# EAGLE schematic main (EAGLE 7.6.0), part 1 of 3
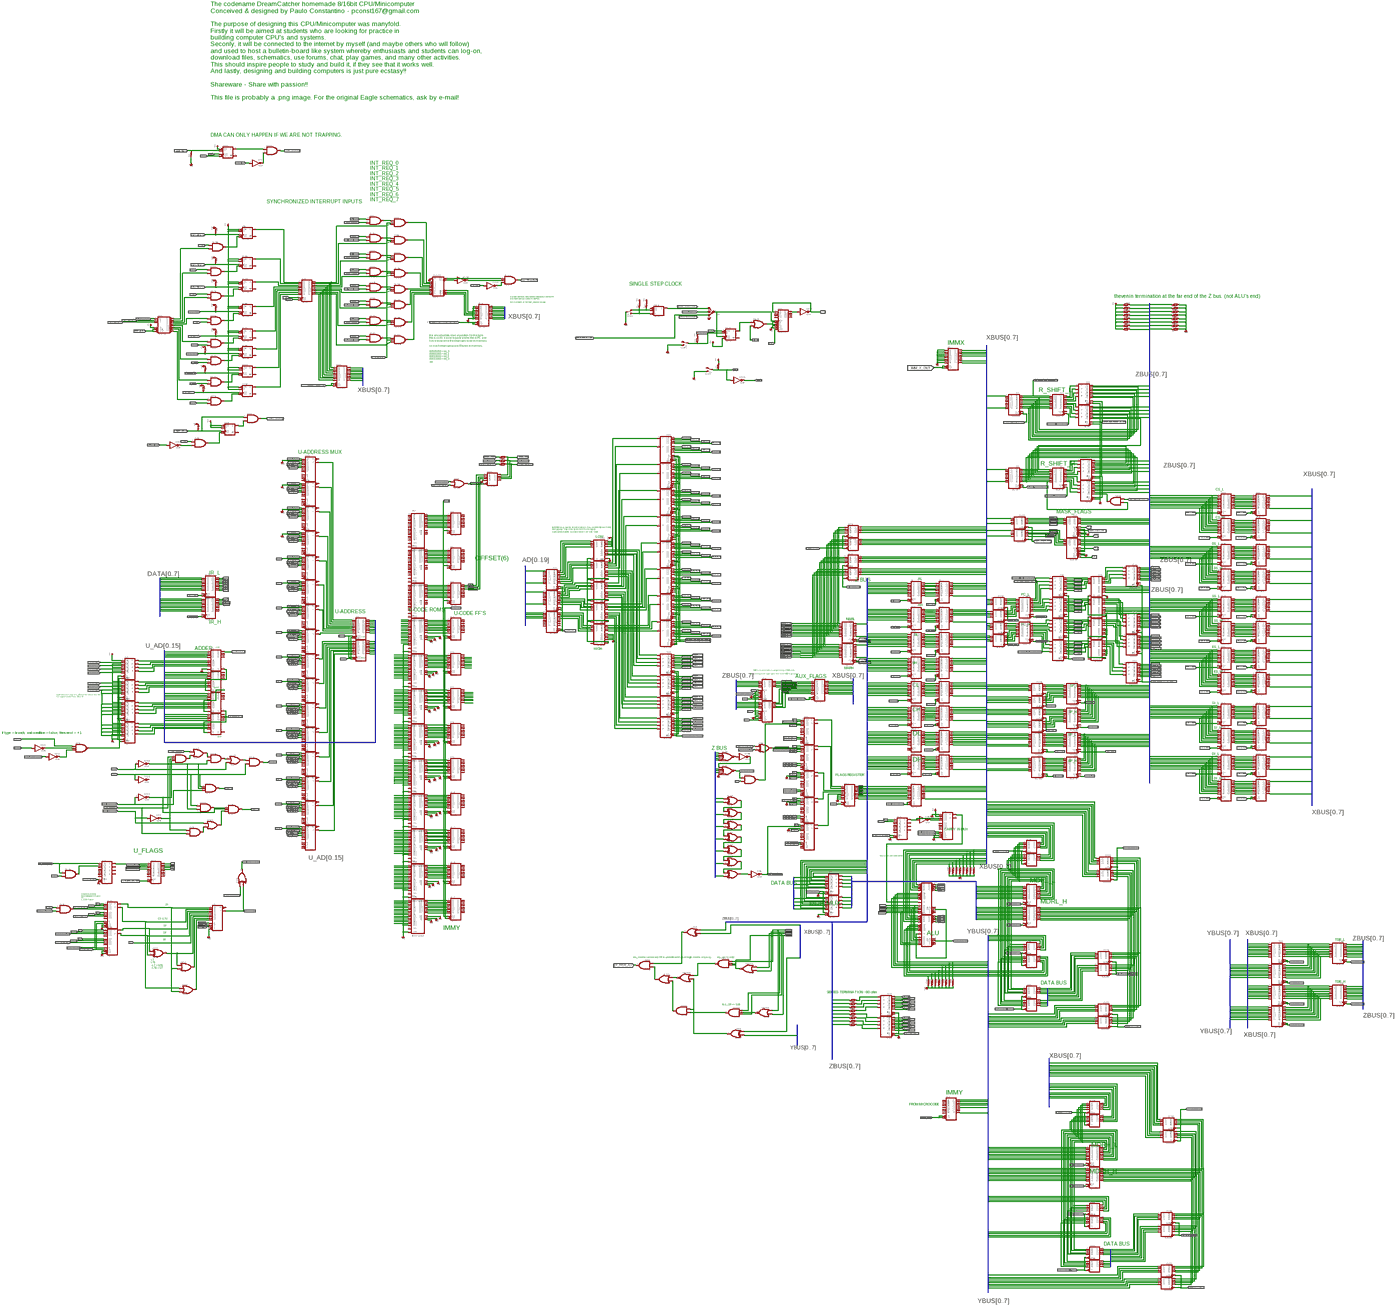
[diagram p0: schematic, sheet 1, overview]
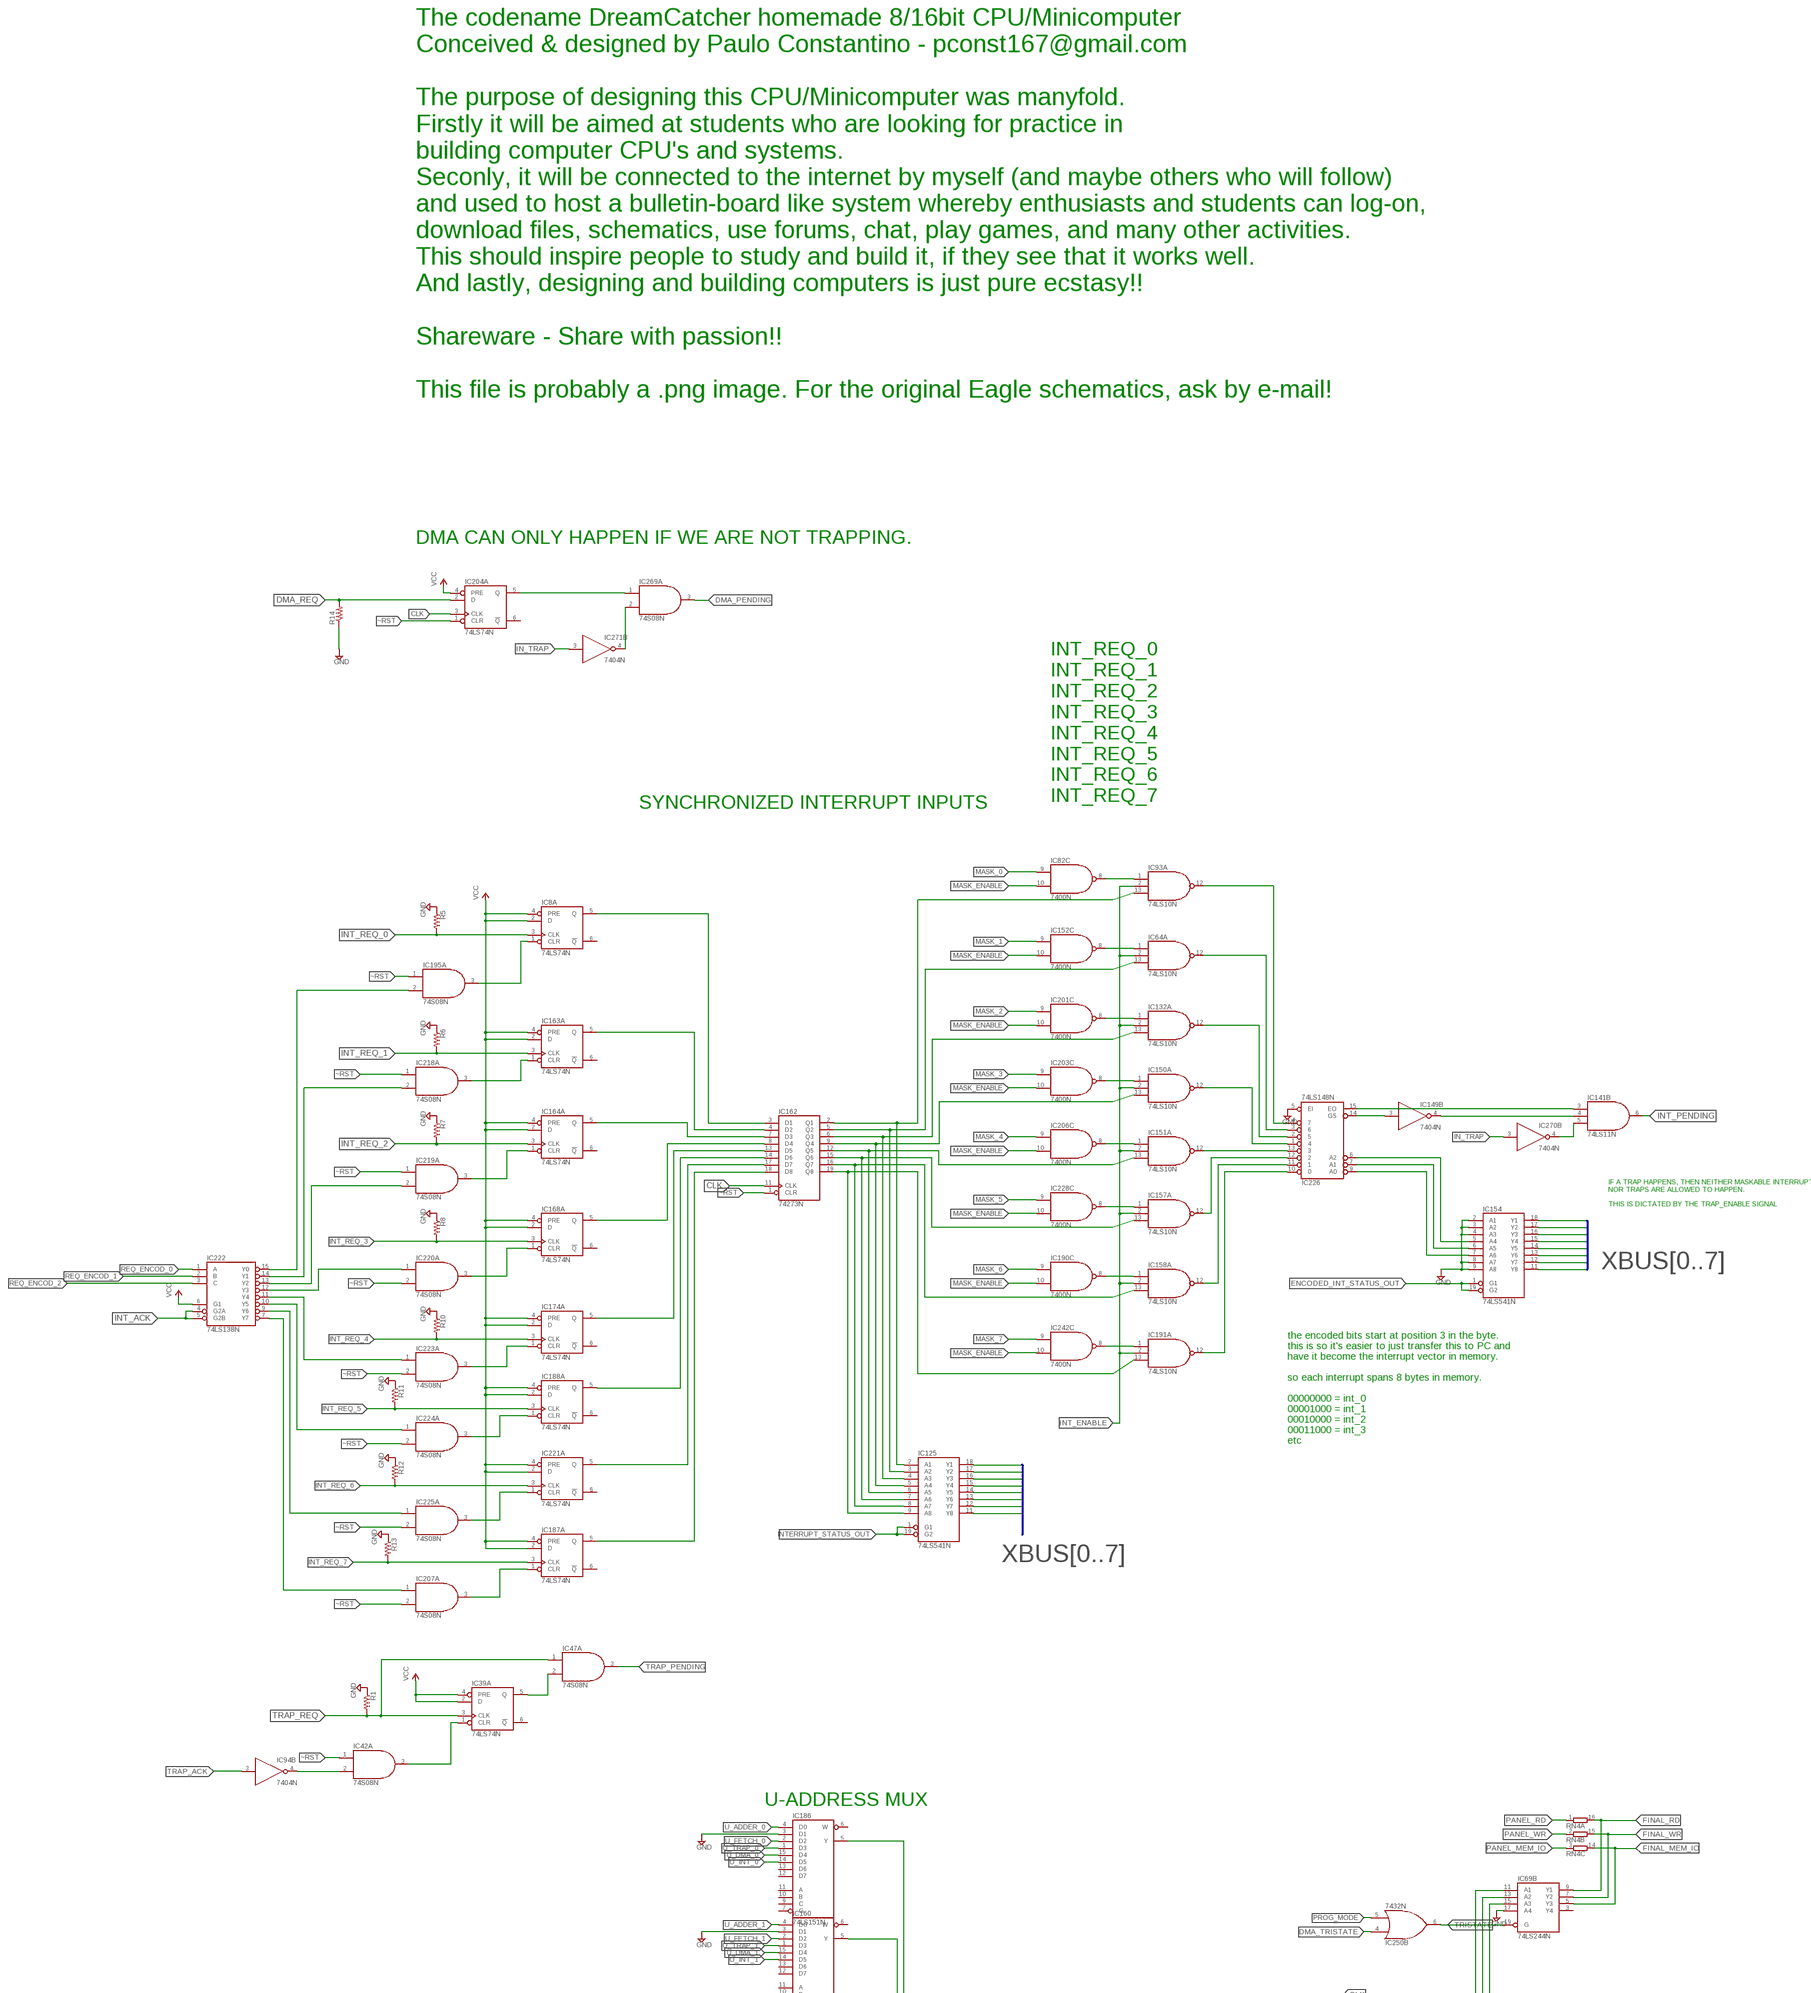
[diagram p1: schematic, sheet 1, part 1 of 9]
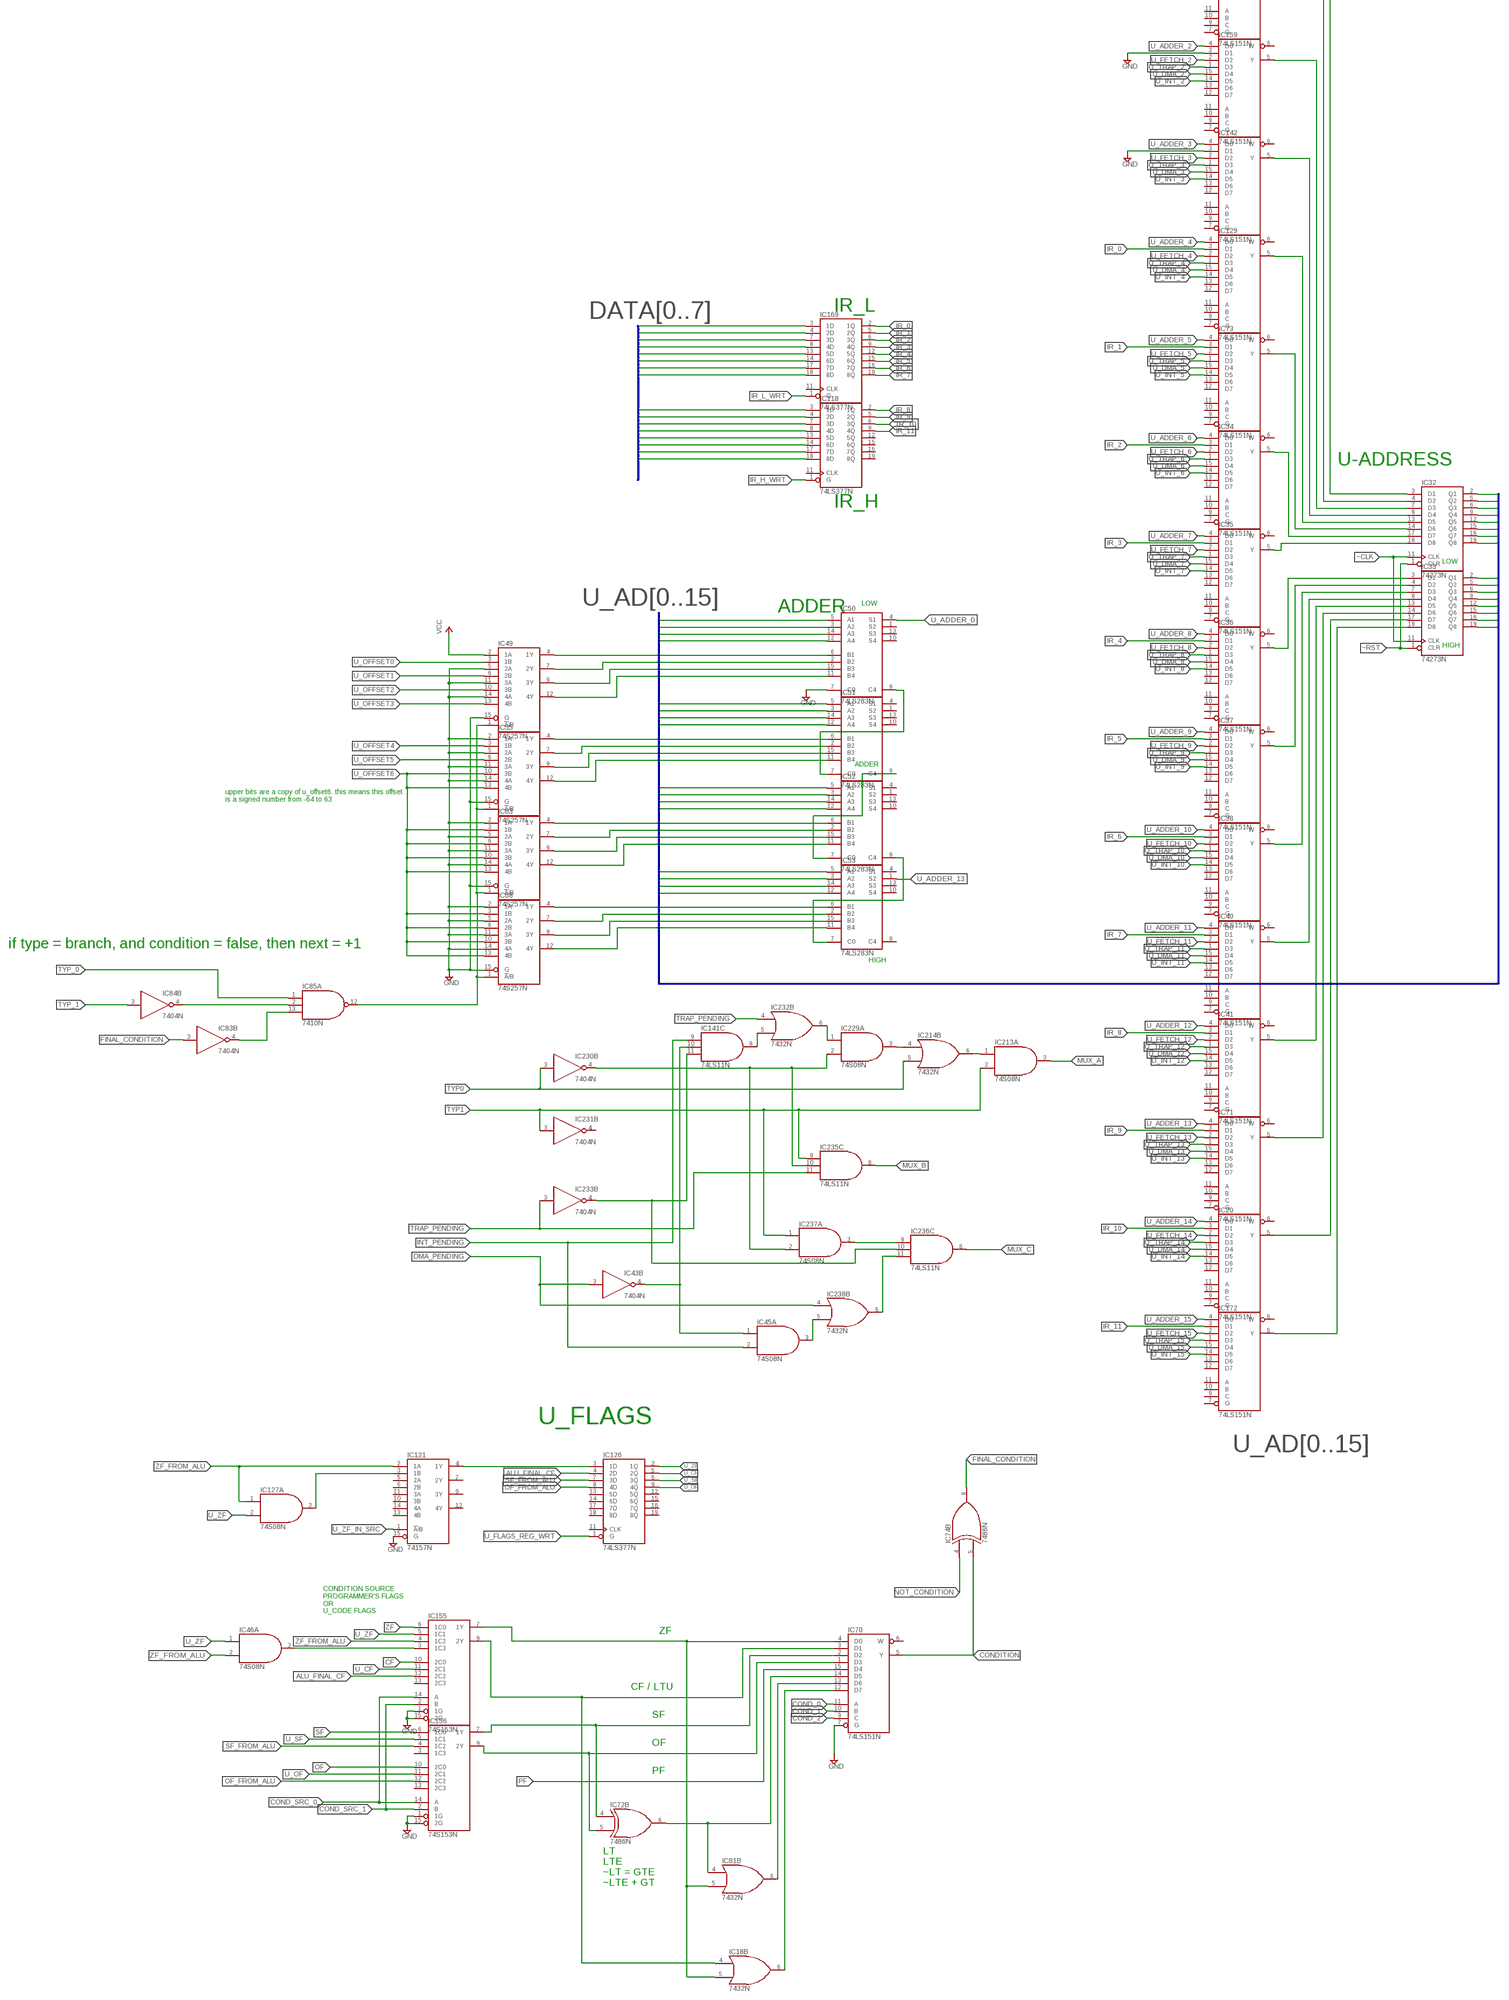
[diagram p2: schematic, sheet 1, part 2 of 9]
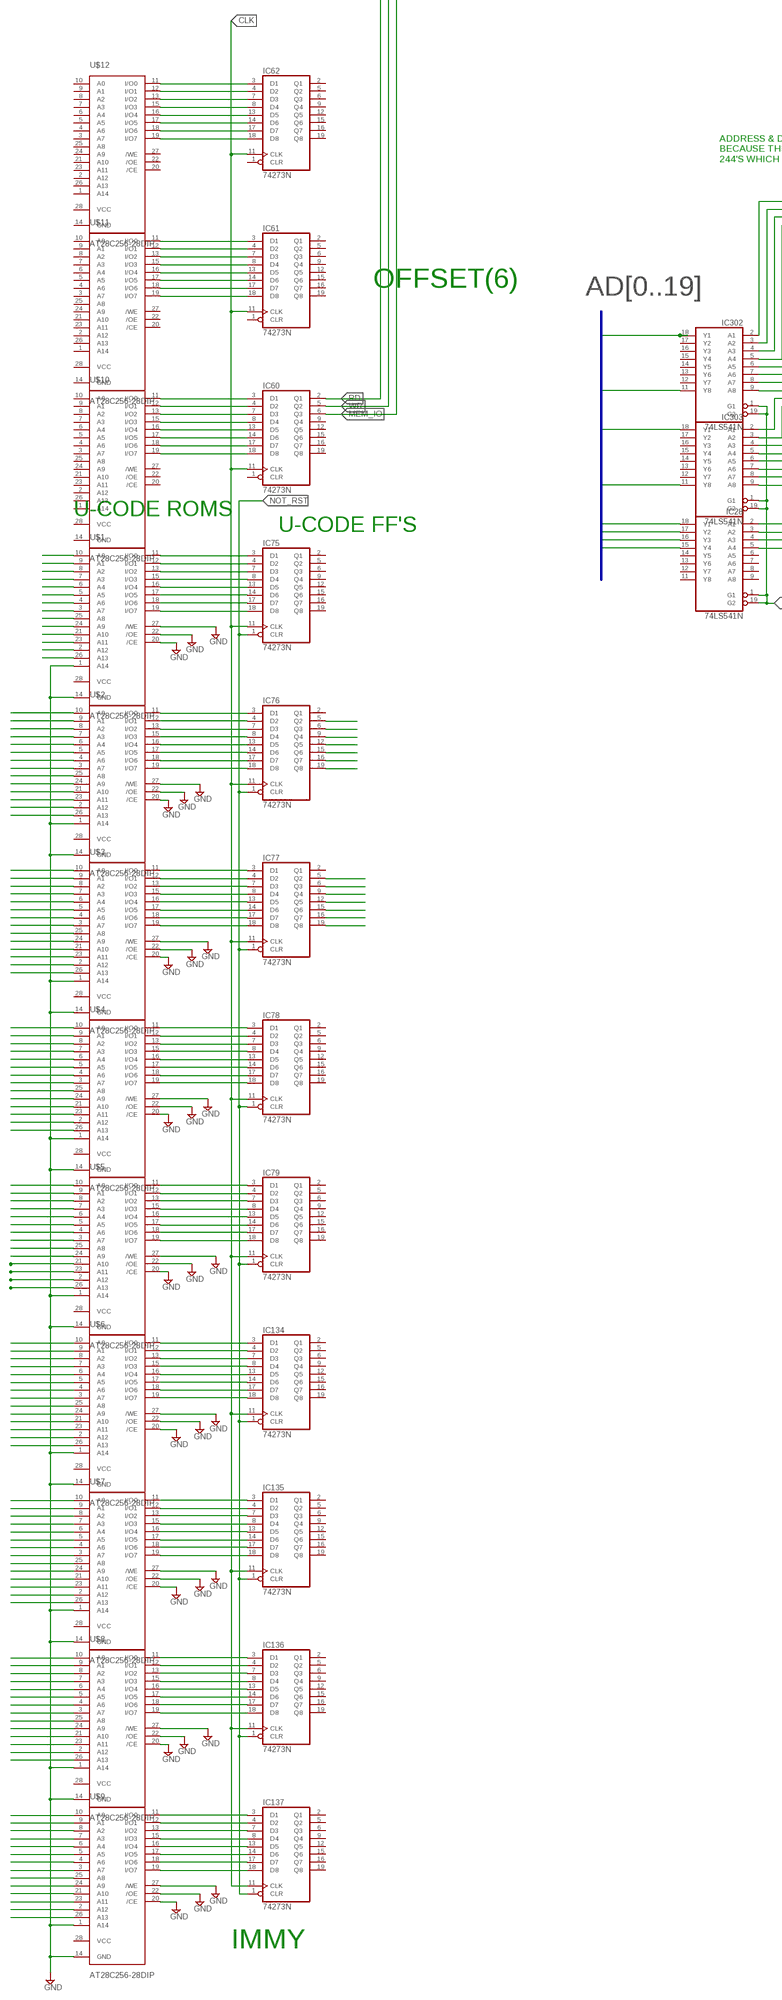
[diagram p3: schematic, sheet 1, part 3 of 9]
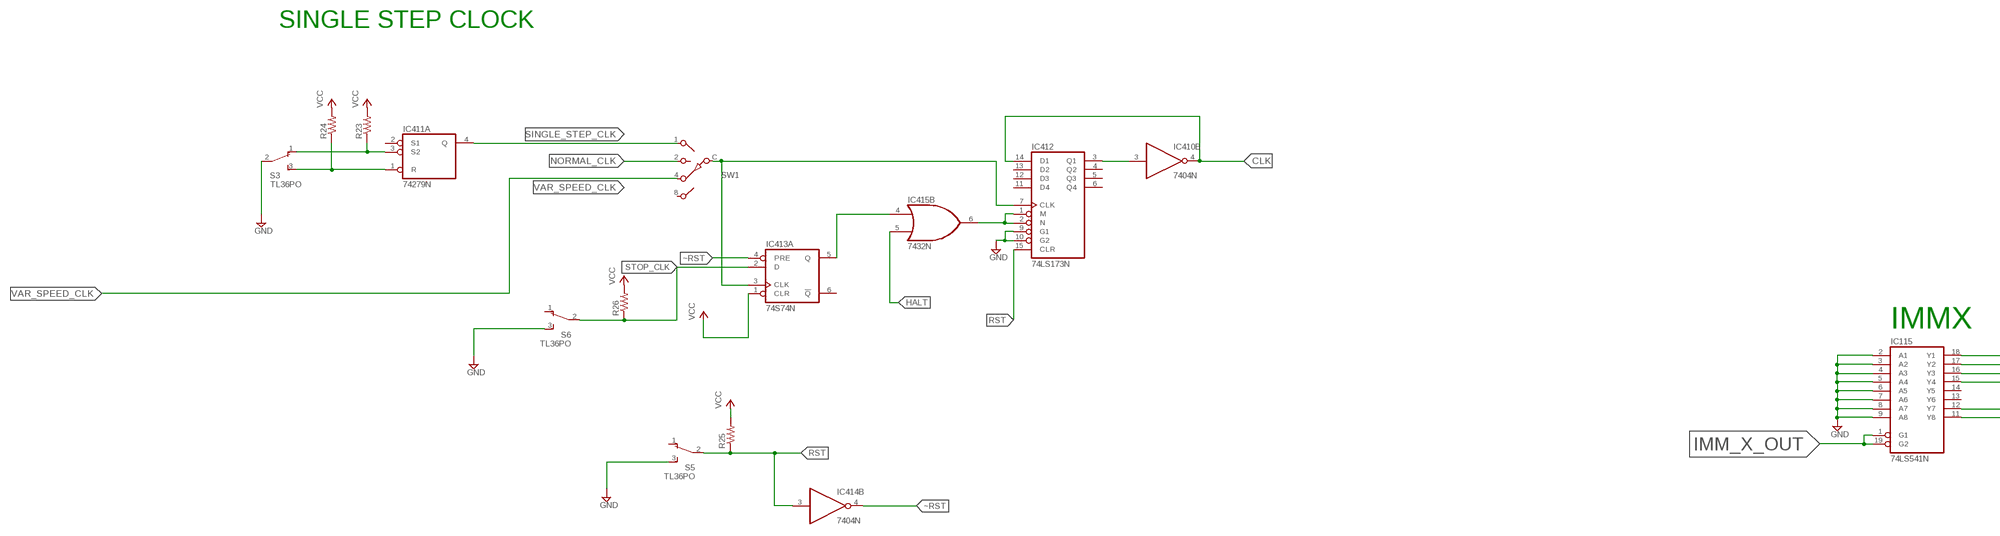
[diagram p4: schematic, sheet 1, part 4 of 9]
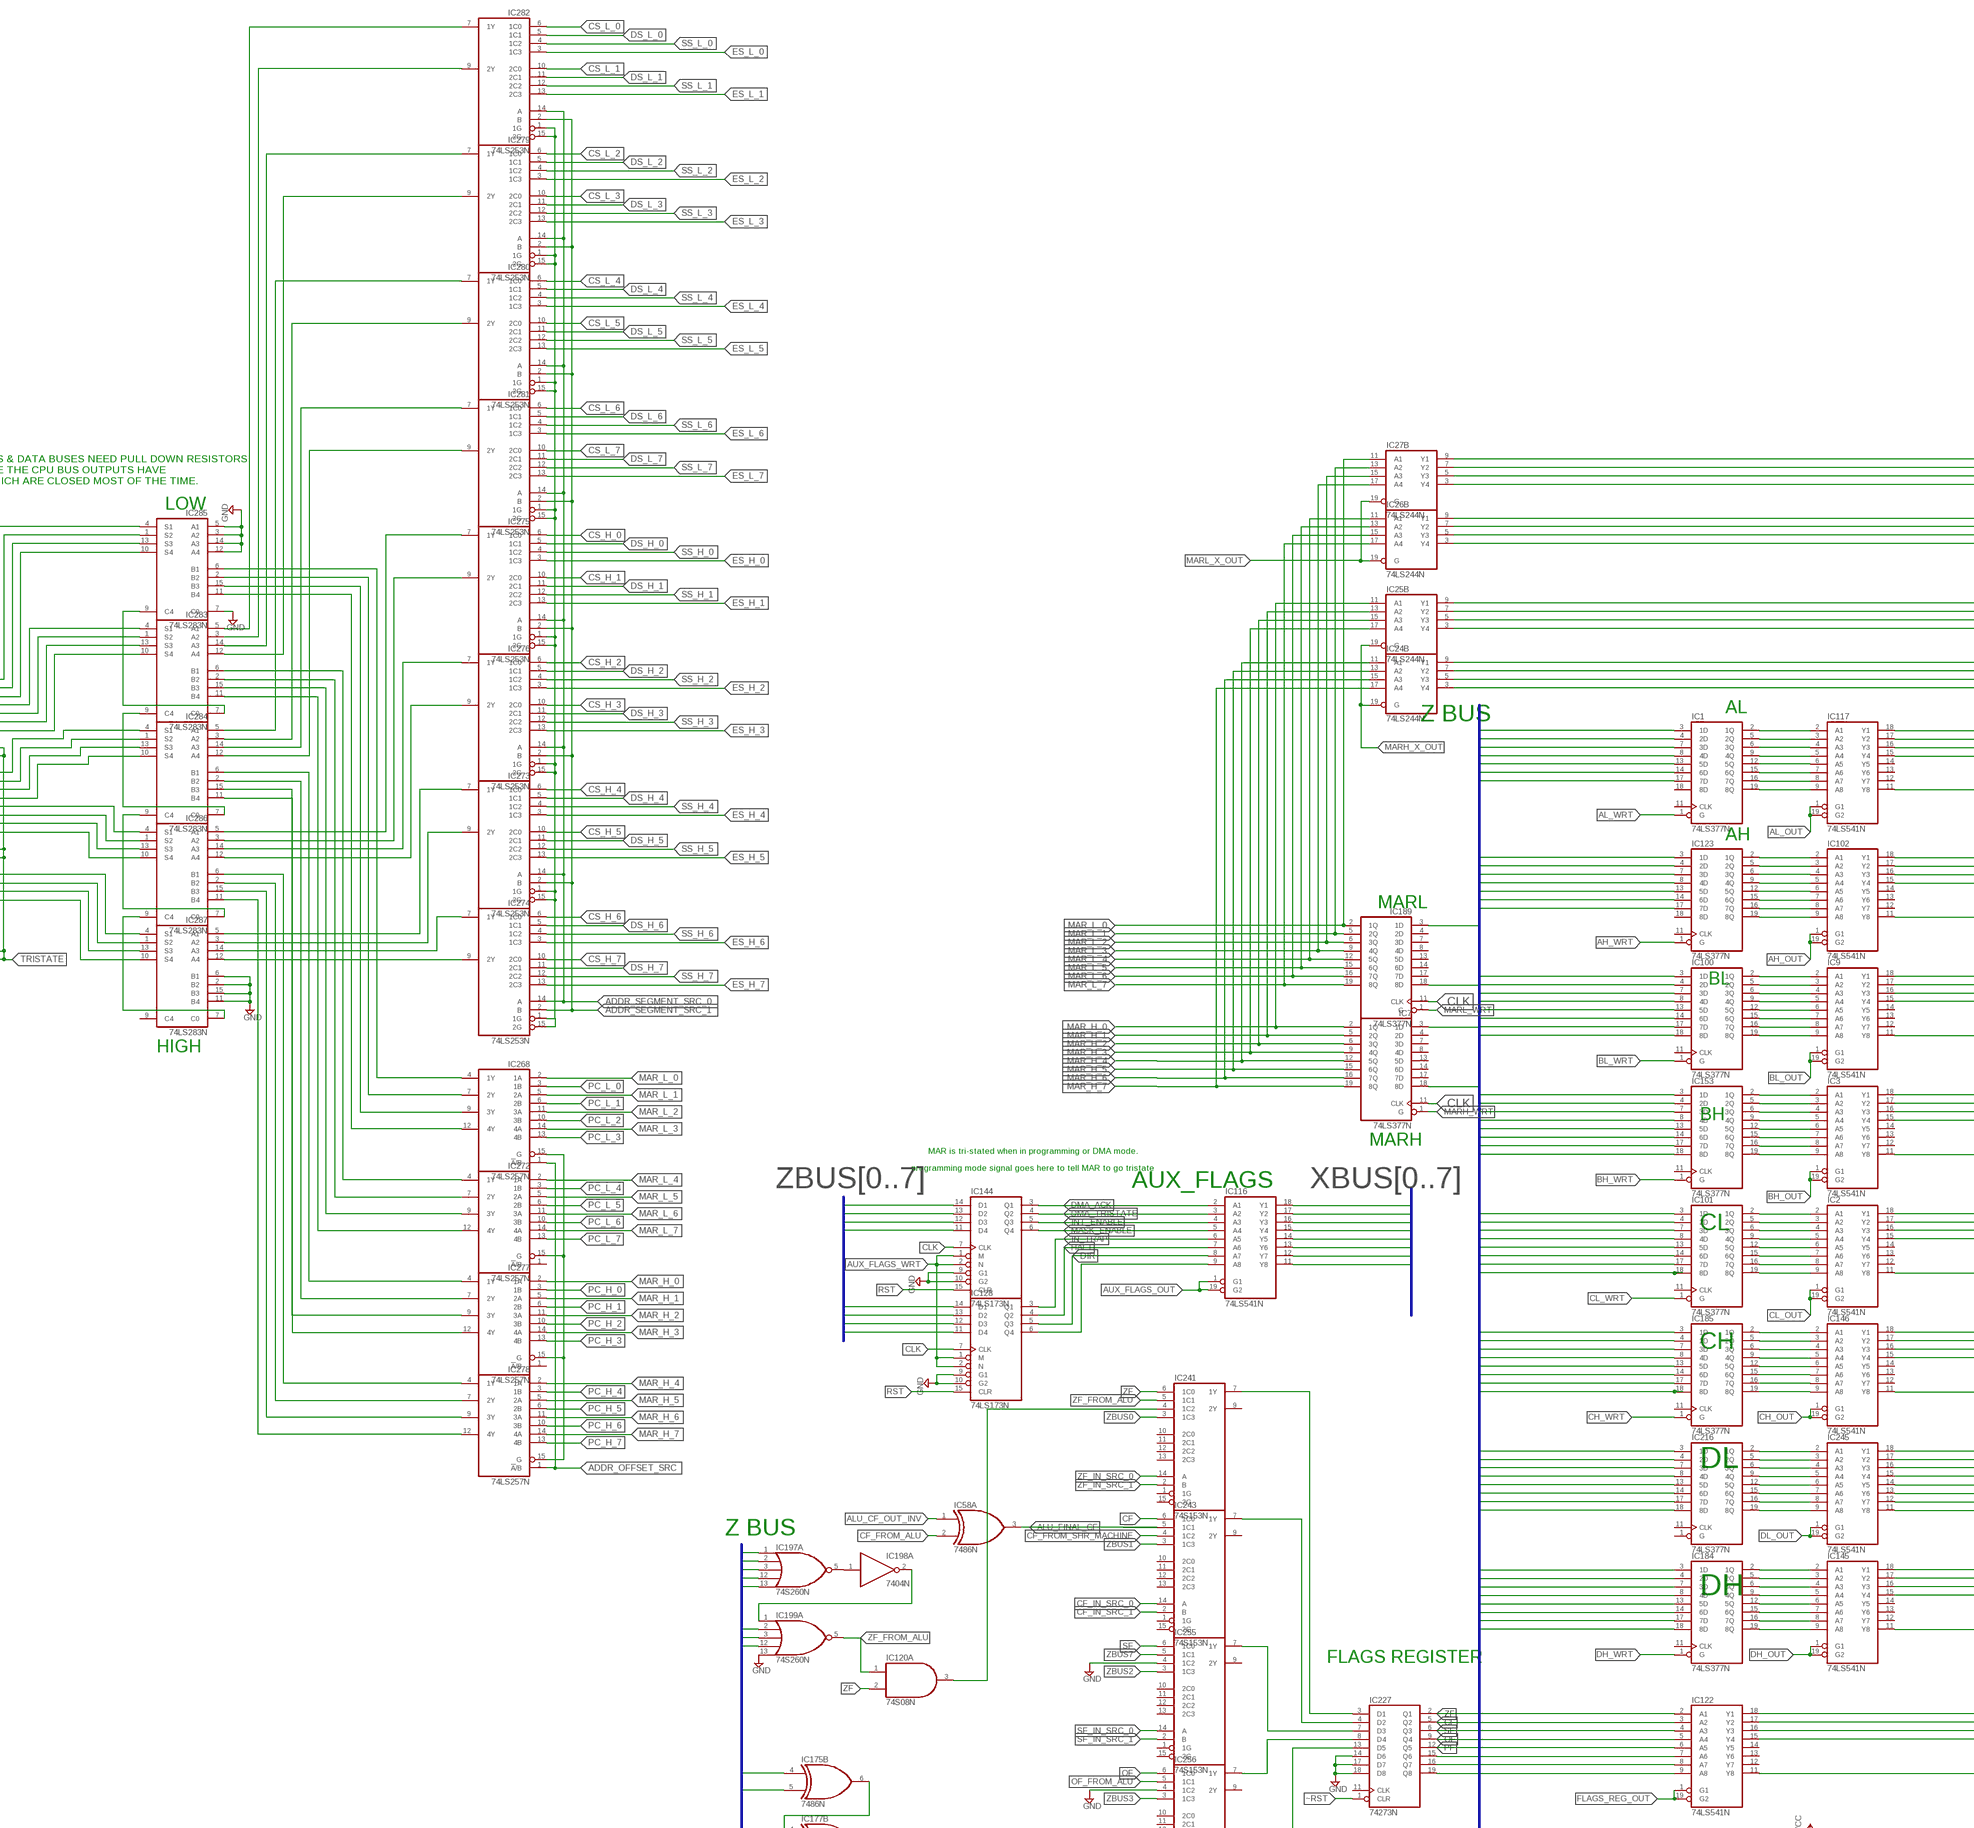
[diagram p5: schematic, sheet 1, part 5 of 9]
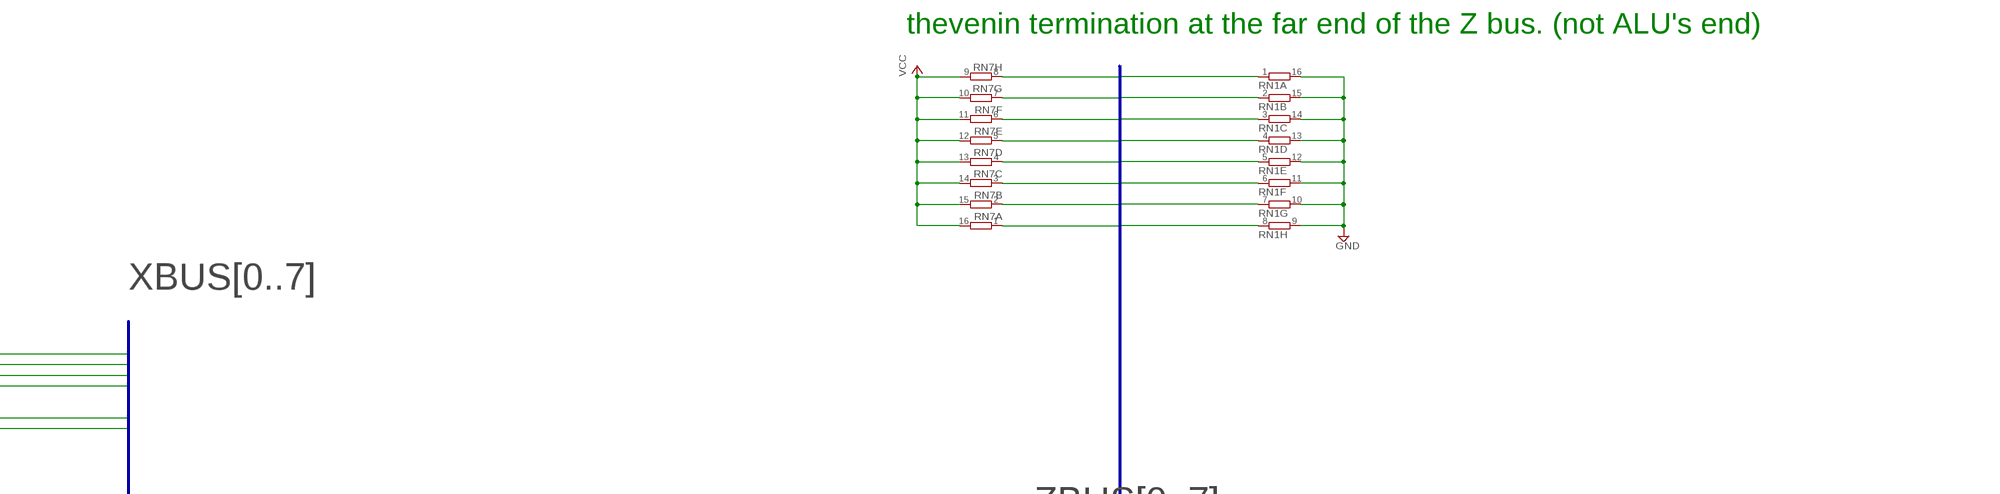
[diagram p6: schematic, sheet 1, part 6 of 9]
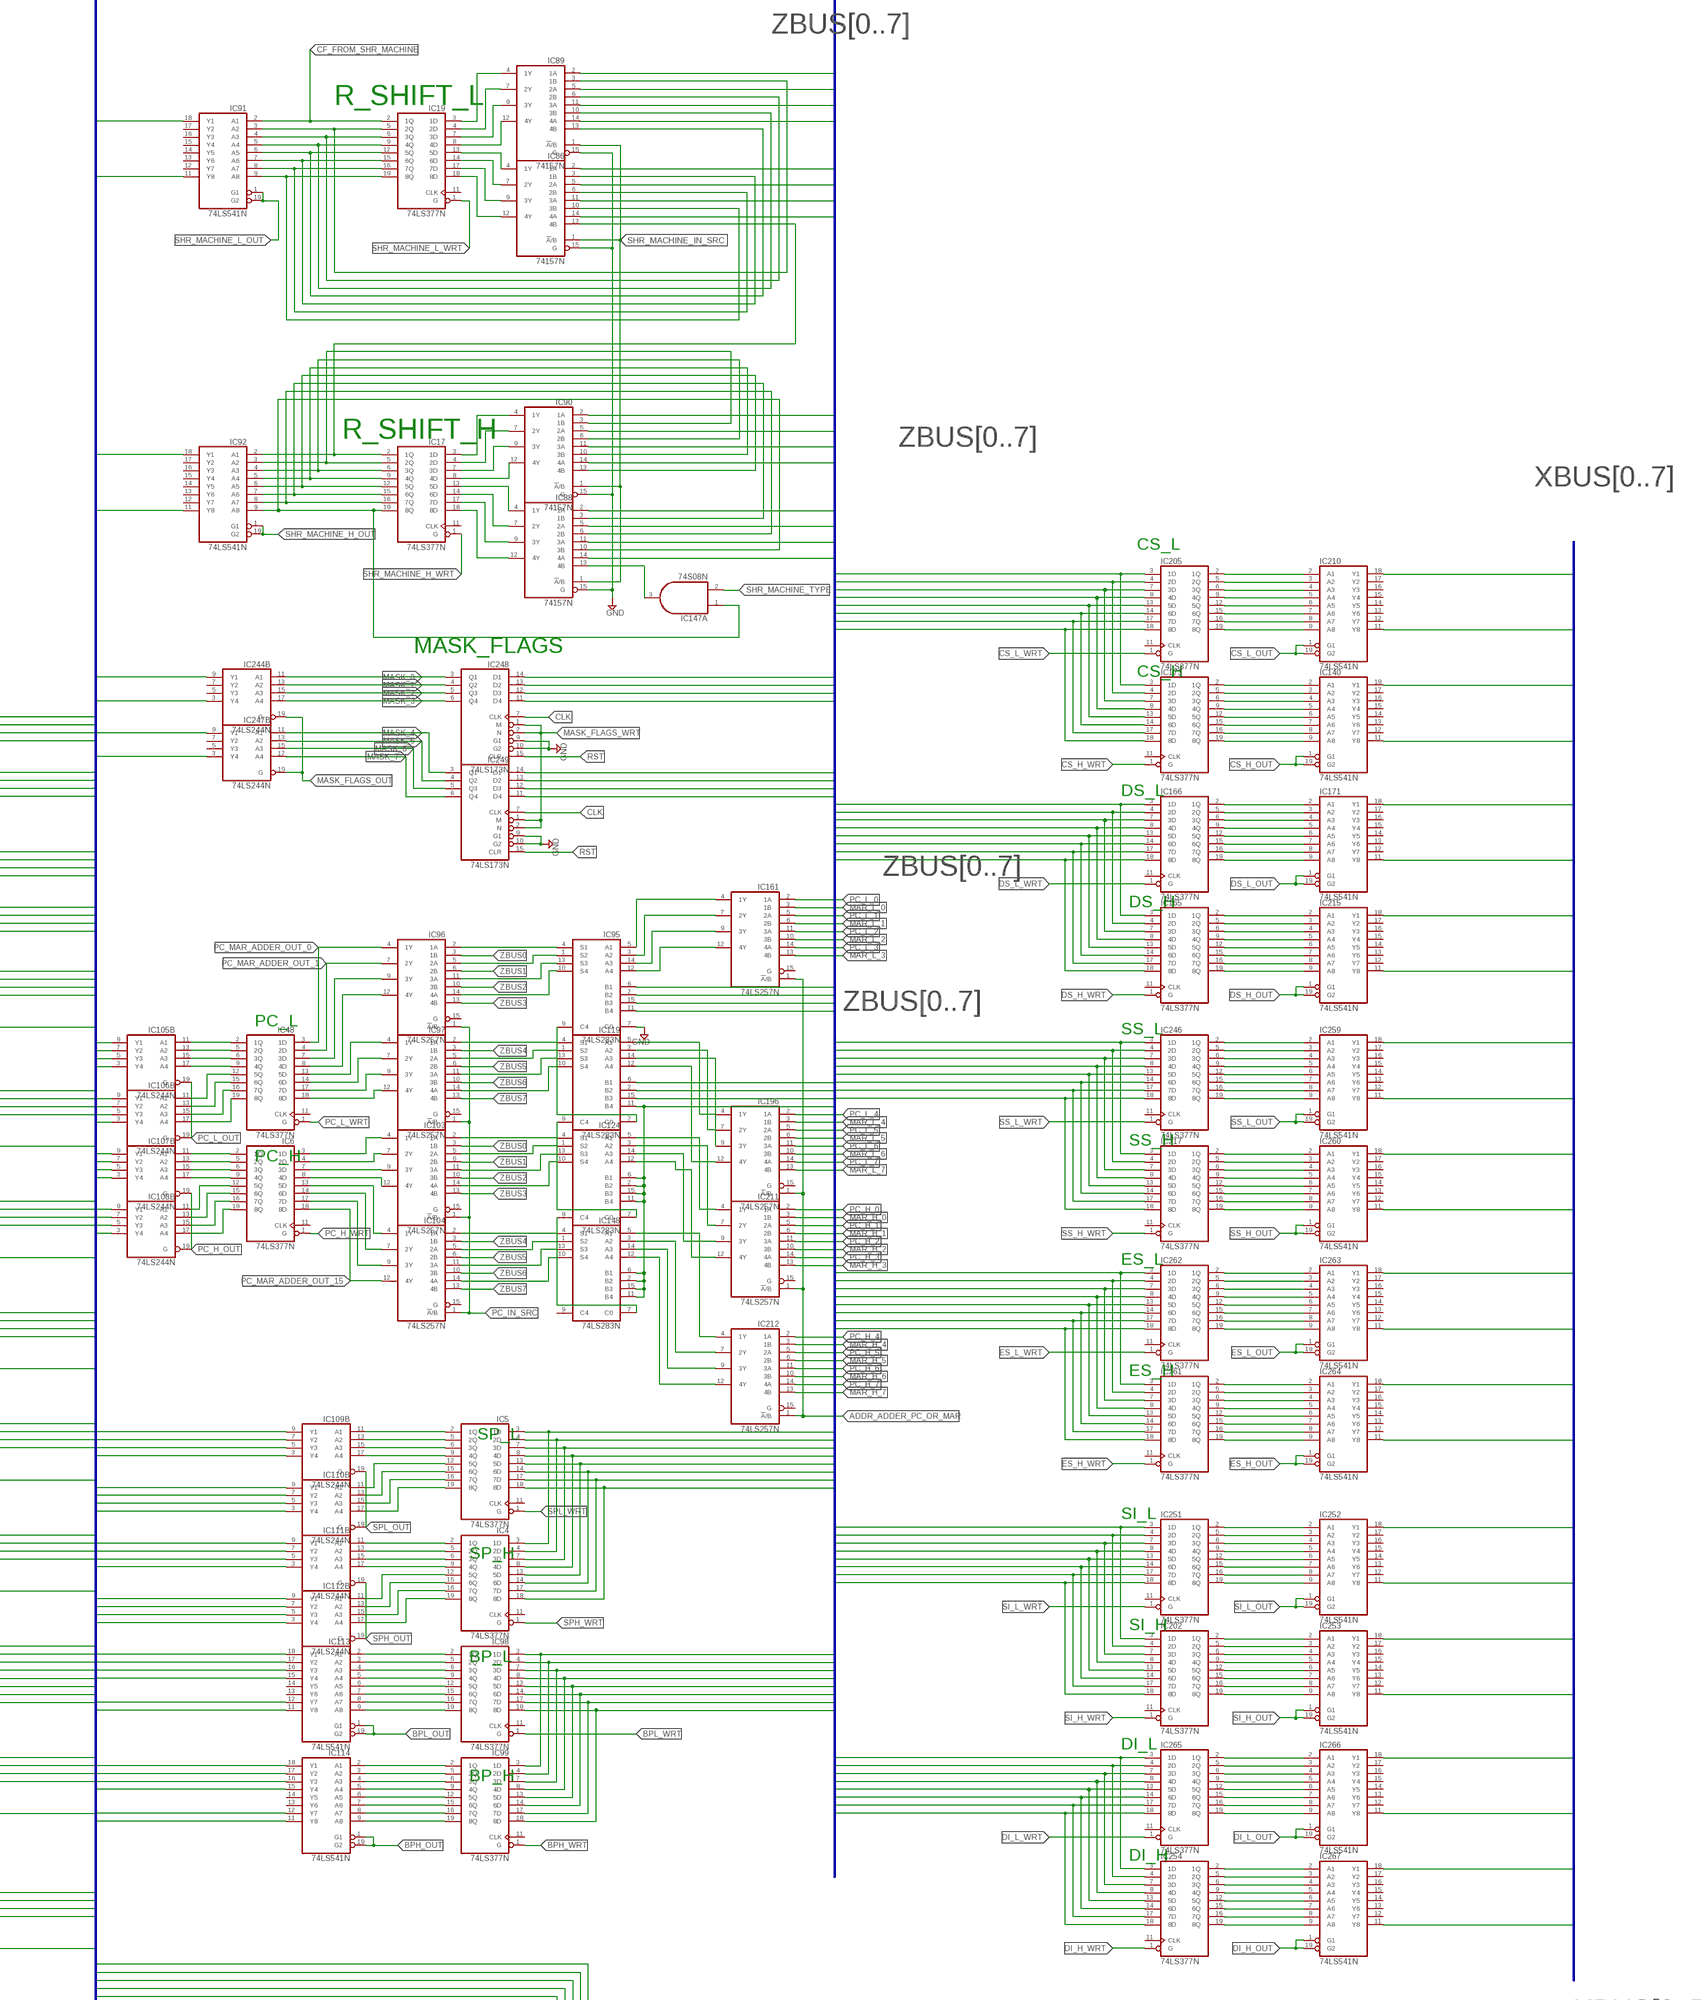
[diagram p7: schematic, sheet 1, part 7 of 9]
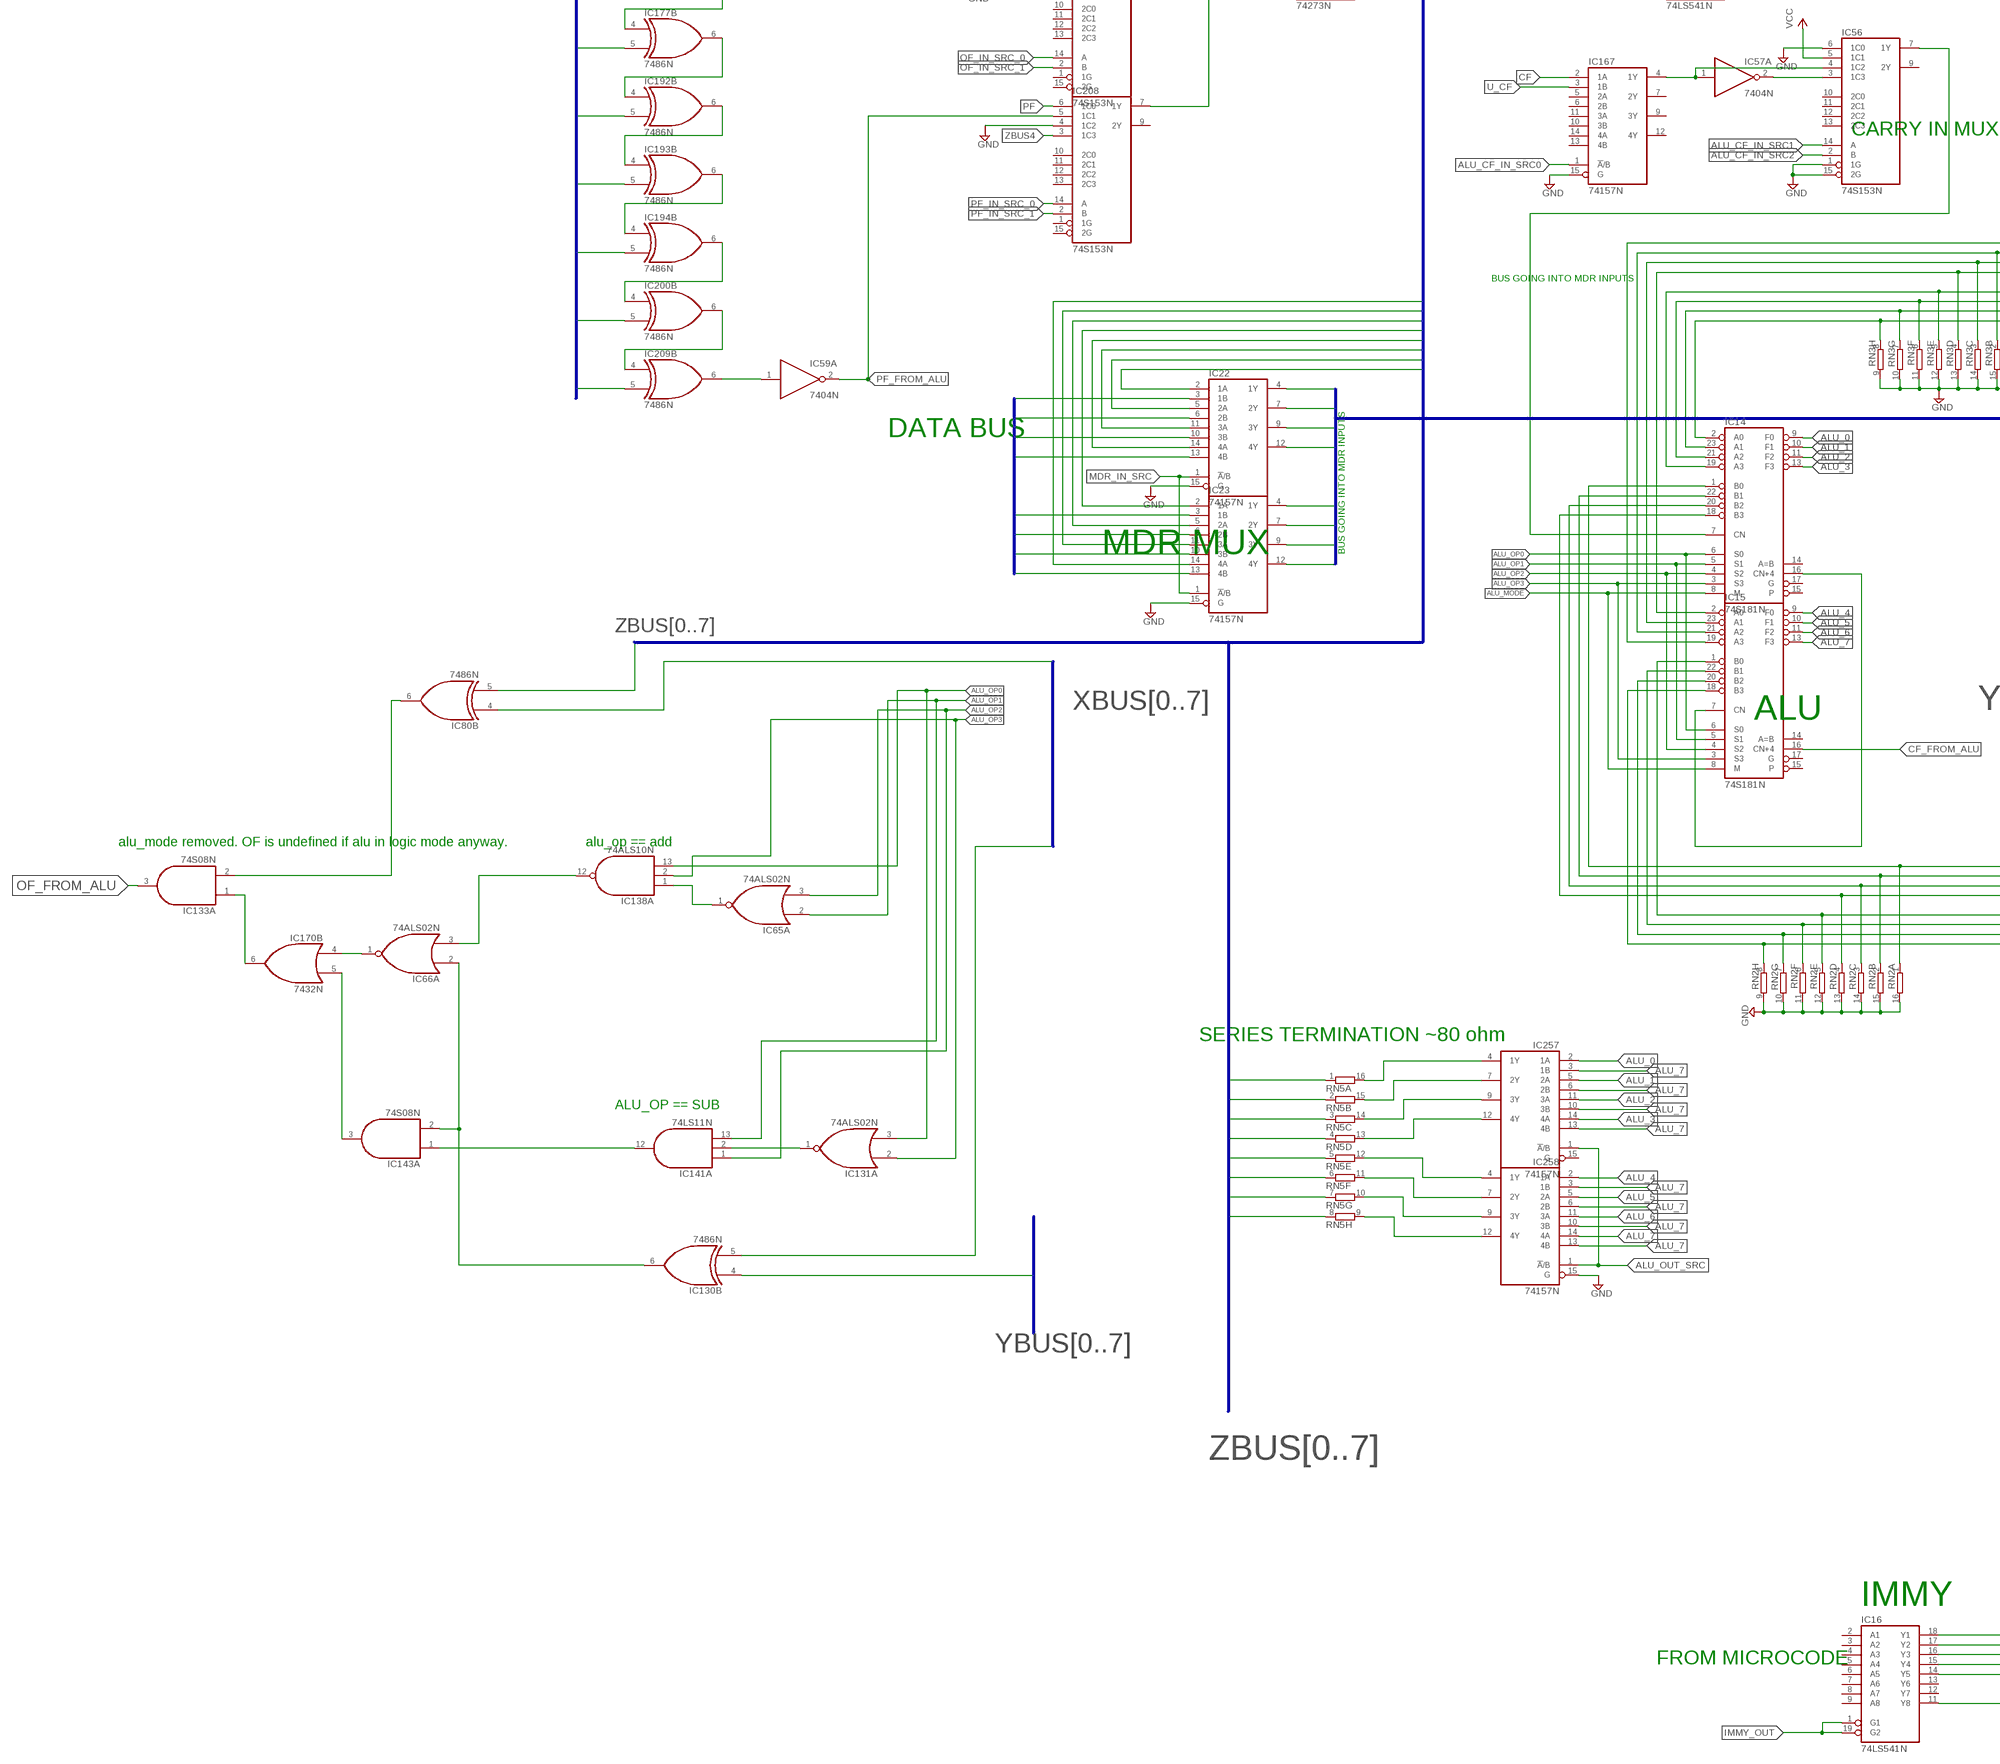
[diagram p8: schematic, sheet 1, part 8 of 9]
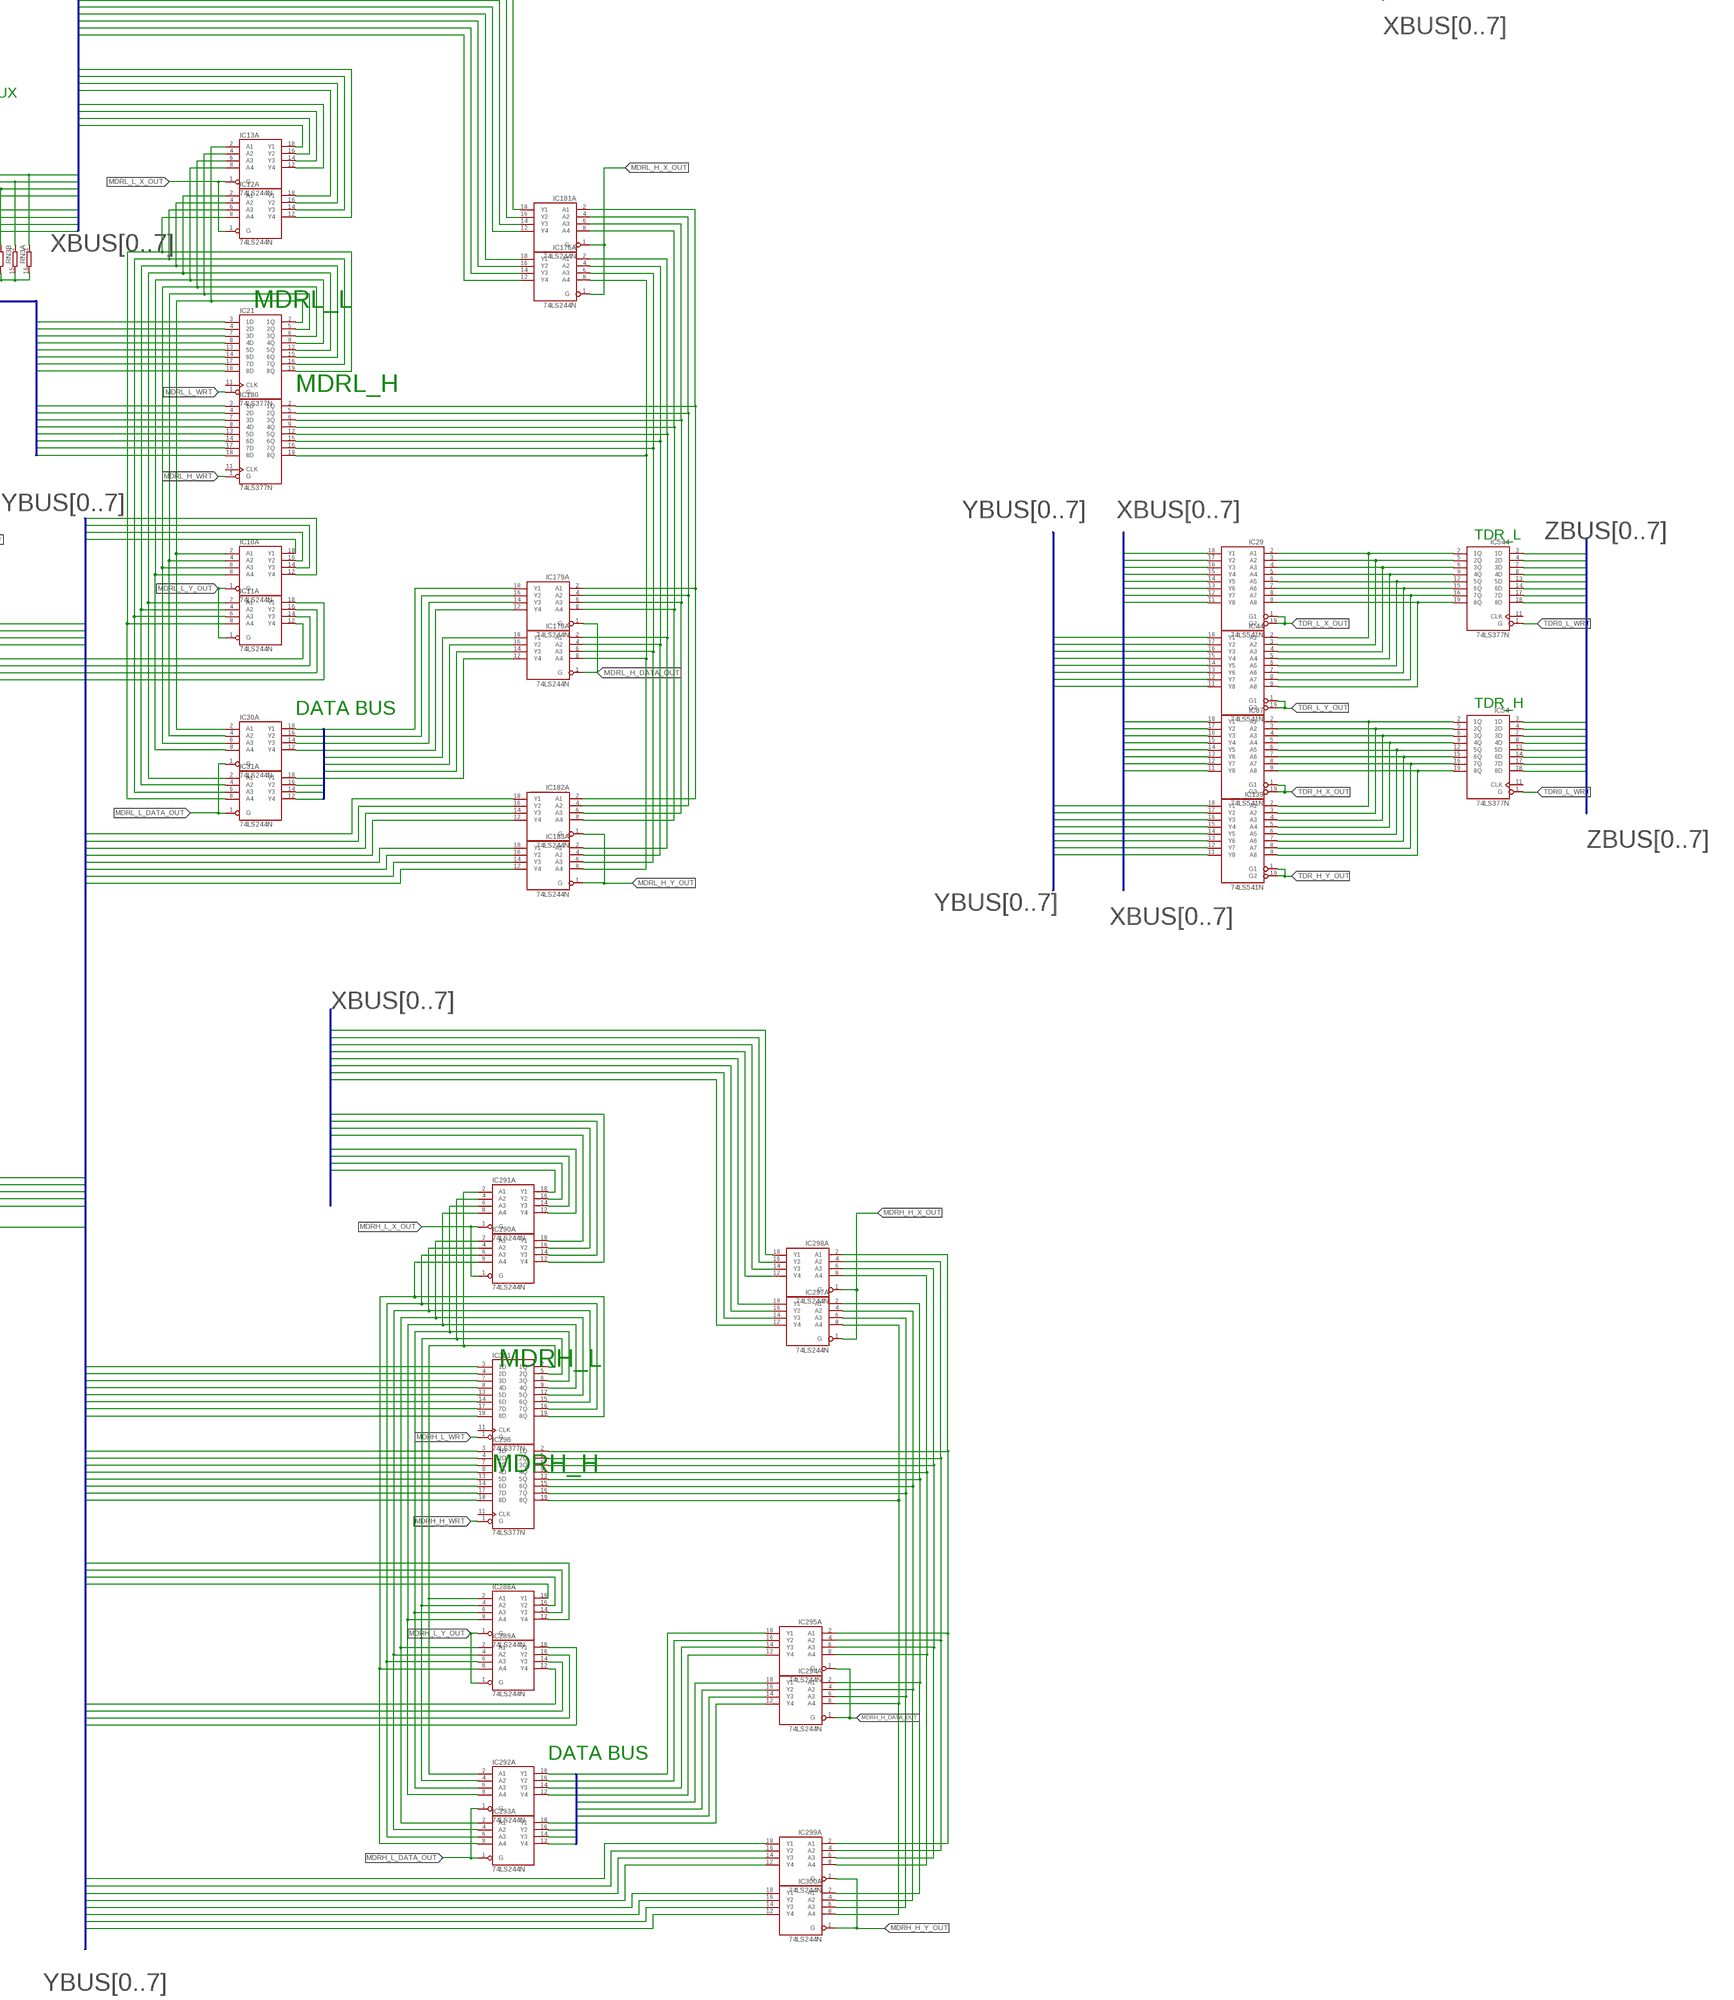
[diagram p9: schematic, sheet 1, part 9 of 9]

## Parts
IC1  74LS377N  [DIL20]
IC2  74LS541N  [DIL20]
IC3  74LS541N  [DIL20]
IC4  74LS377N  [DIL20]
IC5  74LS377N  [DIL20]
IC6  74LS377N  [DIL20]
IC7  74LS377N  [DIL20]
IC8  74LS74N  [DIL14]
IC9  74LS541N  [DIL20]
IC10  74LS244N  [DIL20]
IC11  74LS244N  [DIL20]
IC12  74LS244N  [DIL20]
IC13  74LS244N  [DIL20]
IC14  74S181N  [DIL24-6]
IC15  74S181N  [DIL24-6]
IC16  74LS541N  [DIL20]
IC17  74LS377N  [DIL20]
IC18  7432N  [DIL14]
IC19  74LS377N  [DIL20]
IC20  74LS151N  [DIL16]
IC21  74LS377N  [DIL20]
IC22  74157N  [DIL16]
IC23  74157N  [DIL16]
IC24  74LS244N  [DIL20]
IC25  74LS244N  [DIL20]
IC26  74LS244N  [DIL20]
IC27  74LS244N  [DIL20]
IC28  74LS541N  [DIL20]
IC29  74LS541N  [DIL20]
IC30  74LS244N  [DIL20]
IC31  74LS244N  [DIL20]
IC32  74273N  [DIL20]
IC33  74273N  [DIL20]
IC34  74LS151N  [DIL16]
IC35  74LS151N  [DIL16]
IC36  74LS151N  [DIL16]
IC37  74LS151N  [DIL16]
IC38  74LS151N  [DIL16]
IC39  74LS74N  [DIL14]
IC40  74LS151N  [DIL16]
IC41  74LS151N  [DIL16]
IC42  74S08N  [DIL14]
IC43  7404N  [DIL14]
IC44  74LS541N  [DIL20]
IC45  74S08N  [DIL14]
IC46  74S08N  [DIL14]
IC47  74S08N  [DIL14]
IC48  74LS377N  [DIL20]
IC49  74S257N  [DIL16]
IC50  74LS283N  [DIL16]
IC51  74LS283N  [DIL16]
IC52  74LS283N  [DIL16]
IC53  74LS283N  [DIL16]
IC54  74LS377N  [DIL20]
IC55  74S257N  [DIL16]
IC56  74S153N  [DIL16]
IC57  7404N  [DIL14]
IC58  7486N  [DIL14]
IC59  7404N  [DIL14]
IC60  74273N  [DIL20]
IC61  74273N  [DIL20]
IC62  74273N  [DIL20]
IC63  74S257N  [DIL16]
IC64  74LS10N  [DIL14]
IC65  74ALS02N  [DIL14]
IC66  74ALS02N  [DIL14]
IC68  74S257N  [DIL16]
IC69  74LS244N  [DIL20]
IC70  74LS151N  [DIL16]
IC71  74LS151N  [DIL16]
IC72  7486N  [DIL14]
IC73  74LS151N  [DIL16]
IC74  7486N  [DIL14]
IC75  74273N  [DIL20]
IC76  74273N  [DIL20]
IC77  74273N  [DIL20]
IC78  74273N  [DIL20]
IC79  74273N  [DIL20]
IC80  7486N  [DIL14]
IC81  7432N  [DIL14]
IC82  7400N  [DIL14]
IC83  7404N  [DIL14]
IC84  7404N  [DIL14]
IC85  7410N  [DIL14]
IC86  74157N  [DIL16]
IC87  74LS541N  [DIL20]
IC88  74157N  [DIL16]
IC89  74157N  [DIL16]
IC90  74157N  [DIL16]
IC91  74LS541N  [DIL20]
IC92  74LS541N  [DIL20]
IC93  74LS10N  [DIL14]
IC94  7404N  [DIL14]
IC95  74LS283N  [DIL16]
IC96  74LS257N  [DIL16]
IC97  74LS257N  [DIL16]
IC98  74LS377N  [DIL20]
IC99  74LS377N  [DIL20]
IC100  74LS377N  [DIL20]
IC101  74LS377N  [DIL20]
IC102  74LS541N  [DIL20]
IC103  74LS257N  [DIL16]
IC104  74LS257N  [DIL16]
IC105  74LS244N  [DIL20]
IC106  74LS244N  [DIL20]
IC107  74LS244N  [DIL20]
IC108  74LS244N  [DIL20]
IC109  74LS244N  [DIL20]
IC110  74LS244N  [DIL20]
IC111  74LS244N  [DIL20]
IC112  74LS244N  [DIL20]
IC113  74LS541N  [DIL20]
IC114  74LS541N  [DIL20]
IC115  74LS541N  [DIL20]
IC116  74LS541N  [DIL20]
IC117  74LS541N  [DIL20]
IC118  74LS377N  [DIL20]
IC119  74LS283N  [DIL16]
IC120  74S08N  [DIL14]
IC121  74157N  [DIL16]
IC122  74LS541N  [DIL20]
IC123  74LS377N  [DIL20]
IC124  74LS283N  [DIL16]
IC125  74LS541N  [DIL20]
IC126  74LS377N  [DIL20]
IC127  74S08N  [DIL14]
IC128  74LS173N  [DIL16]
IC129  74LS151N  [DIL16]
IC130  7486N  [DIL14]
IC131  74ALS02N  [DIL14]
IC132  74LS10N  [DIL14]
IC133  74S08N  [DIL14]
IC134  74273N  [DIL20]
IC135  74273N  [DIL20]
IC136  74273N  [DIL20]
IC137  74273N  [DIL20]
IC138  74ALS10N  [DIL14]
IC139  74LS541N  [DIL20]
IC140  74LS541N  [DIL20]
IC141  74LS11N  [DIL14]
IC142  74LS151N  [DIL16]
IC143  74S08N  [DIL14]
IC144  74LS173N  [DIL16]
IC145  74LS541N  [DIL20]
IC146  74LS541N  [DIL20]
IC147  74S08N  [DIL14]
IC148  74LS283N  [DIL16]
IC149  7404N  [DIL14]
IC150  74LS10N  [DIL14]
IC151  74LS10N  [DIL14]
IC152  7400N  [DIL14]
IC153  74LS377N  [DIL20]
IC154  74LS541N  [DIL20]
IC155  74S153N  [DIL16]
IC156  74S153N  [DIL16]
IC157  74LS10N  [DIL14]
IC158  74LS10N  [DIL14]
IC159  74LS151N  [DIL16]
IC160  74LS151N  [DIL16]
IC161  74LS257N  [DIL16]
IC162  74273N  [DIL20]
IC163  74LS74N  [DIL14]
IC164  74LS74N  [DIL14]
IC165  74LS377N  [DIL20]
IC166  74LS377N  [DIL20]
IC167  74157N  [DIL16]
IC168  74LS74N  [DIL14]
IC169  74LS377N  [DIL20]
IC170  7432N  [DIL14]
IC171  74LS541N  [DIL20]
IC172  74LS151N  [DIL16]
IC173  74LS377N  [DIL20]
IC174  74LS74N  [DIL14]
IC175  7486N  [DIL14]
IC176  74LS244N  [DIL20]
IC177  7486N  [DIL14]
IC178  74LS244N  [DIL20]
IC179  74LS244N  [DIL20]
IC180  74LS377N  [DIL20]
IC181  74LS244N  [DIL20]
IC182  74LS244N  [DIL20]
IC183  74LS244N  [DIL20]
IC184  74LS377N  [DIL20]
IC185  74LS377N  [DIL20]
IC186  74LS151N  [DIL16]
IC187  74LS74N  [DIL14]
IC188  74LS74N  [DIL14]
IC189  74LS377N  [DIL20]
IC190  7400N  [DIL14]
IC191  74LS10N  [DIL14]
IC192  7486N  [DIL14]
IC193  7486N  [DIL14]
IC194  7486N  [DIL14]
IC195  74S08N  [DIL14]
IC196  74LS257N  [DIL16]
IC197  74S260N  [DIL14]
IC198  7404N  [DIL14]
IC199  74S260N  [DIL14]
IC200  7486N  [DIL14]
IC201  7400N  [DIL14]
IC202  74LS377N  [DIL20]
IC203  7400N  [DIL14]
IC204  74LS74N  [DIL14]
IC205  74LS377N  [DIL20]
IC206  7400N  [DIL14]
IC207  74S08N  [DIL14]
IC208  74S153N  [DIL16]
IC209  7486N  [DIL14]
IC210  74LS541N  [DIL20]
IC211  74LS257N  [DIL16]
IC212  74LS257N  [DIL16]
IC213  74S08N  [DIL14]
IC214  7432N  [DIL14]
IC215  74LS541N  [DIL20]
IC216  74LS377N  [DIL20]
IC217  74LS377N  [DIL20]
IC218  74S08N  [DIL14]
IC219  74S08N  [DIL14]
IC220  74S08N  [DIL14]
IC221  74LS74N  [DIL14]
IC222  74LS138N  [DIL16]
IC223  74S08N  [DIL14]
IC224  74S08N  [DIL14]
IC225  74S08N  [DIL14]
IC226  74LS148N  [DIL16]
IC227  74273N  [DIL20]
IC228  7400N  [DIL14]
IC229  74S08N  [DIL14]
IC230  7404N  [DIL14]
IC231  7404N  [DIL14]
IC232  7432N  [DIL14]
IC233  7404N  [DIL14]
IC235  74LS11N  [DIL14]
IC236  74LS11N  [DIL14]
IC237  74S08N  [DIL14]
IC238  7432N  [DIL14]
IC241  74S153N  [DIL16]
IC242  7400N  [DIL14]
IC243  74S153N  [DIL16]
IC244  74LS244N  [DIL20]
IC245  74LS541N  [DIL20]
IC246  74LS377N  [DIL20]
IC247  74LS244N  [DIL20]
IC248  74LS173N  [DIL16]
IC249  74LS173N  [DIL16]
IC250  7432N  [DIL14]
IC251  74LS377N  [DIL20]
IC252  74LS541N  [DIL20]
IC253  74LS541N  [DIL20]
IC254  74LS377N  [DIL20]
IC255  74S153N  [DIL16]
IC256  74S153N  [DIL16]
IC257  74157N  [DIL16]
IC258  74157N  [DIL16]
IC259  74LS541N  [DIL20]
IC260  74LS541N  [DIL20]
IC261  74LS377N  [DIL20]
IC262  74LS377N  [DIL20]
IC263  74LS541N  [DIL20]
IC264  74LS541N  [DIL20]
IC265  74LS377N  [DIL20]
IC266  74LS541N  [DIL20]
IC267  74LS541N  [DIL20]
IC268  74LS257N  [DIL16]
IC269  74S08N  [DIL14]
IC270  7404N  [DIL14]
IC271  7404N  [DIL14]
IC272  74LS257N  [DIL16]
IC273  74LS253N  [DIL16]
IC274  74LS253N  [DIL16]
IC275  74LS253N  [DIL16]
IC276  74LS253N  [DIL16]
IC277  74LS257N  [DIL16]
IC278  74LS257N  [DIL16]
IC279  74LS253N  [DIL16]
IC280  74LS253N  [DIL16]
IC281  74LS253N  [DIL16]
IC282  74LS253N  [DIL16]
IC283  74LS283N  [DIL16]
IC284  74LS283N  [DIL16]
IC285  74LS283N  [DIL16]
IC286  74LS283N  [DIL16]
IC287  74LS283N  [DIL16]
IC288  74LS244N  [DIL20]
IC289  74LS244N  [DIL20]
IC290  74LS244N  [DIL20]
IC291  74LS244N  [DIL20]
IC292  74LS244N  [DIL20]
IC293  74LS244N  [DIL20]
IC294  74LS244N  [DIL20]
IC295  74LS244N  [DIL20]
IC296  74LS377N  [DIL20]
IC297  74LS244N  [DIL20]
IC298  74LS244N  [DIL20]
IC299  74LS244N  [DIL20]
IC300  74LS244N  [DIL20]
IC301  74LS377N  [DIL20]
IC302  74LS541N  [DIL20]
IC303  74LS541N  [DIL20]
IC410  7404N  [DIL14]
IC411  74279N  [DIL16]
IC412  74LS173N  [DIL16]
IC413  74S74N  [DIL14]
IC414  7404N  [DIL14]
IC415  7432N  [DIL14]
IC544  74LS377N  [DIL20]
R1  R-US_0204/7  [0204/7]
R5  R-US_0204/7  [0204/7]
R6  R-US_0204/7  [0204/7]
R7  R-US_0204/7  [0204/7]
R8  R-US_0204/7  [0204/7]
R10  R-US_0204/7  [0204/7]
R11  R-US_0204/7  [0204/7]
R12  R-US_0204/7  [0204/7]
R13  R-US_0204/7  [0204/7]
R14  R-US_0204/7  [0204/7]
R23  R-US_0204/2V  [0204V]
R24  R-US_0204/2V  [0204V]
R25  R-US_0204/2V  [0204V]
R26  R-US_0204/2V  [0204V]
RN1  8R-N  [DIL16]
RN2  8R-N  [DIL16]
RN3  8R-N  [DIL16]
RN4  8R-N  [DIL16]
RN5  8R-N  [DIL16]
RN7  8R-N  [DIL16]
S3  TL36PO  [TL3XPO]
S5  TL36PO  [TL3XPO]
S6  TL36PO  [TL3XPO]
SW1  SW-C10  [SW-C10]
U$1  AT28C256-28DIP  [DIL28-6]
U$2  AT28C256-28DIP  [DIL28-6]
U$3  AT28C256-28DIP  [DIL28-6]
U$4  AT28C256-28DIP  [DIL28-6]
U$5  AT28C256-28DIP  [DIL28-6]
U$6  AT28C256-28DIP  [DIL28-6]
U$7  AT28C256-28DIP  [DIL28-6]
U$8  AT28C256-28DIP  [DIL28-6]
U$9  AT28C256-28DIP  [DIL28-6]
U$10  AT28C256-28DIP  [DIL28-6]
U$11  AT28C256-28DIP  [DIL28-6]
U$12  AT28C256-28DIP  [DIL28-6]

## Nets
45435: IC18.5(B:I1) IC70.4(D0) IC81.5(B:I1) IC155.7(1Y)
345345: IC70.2(D2) IC72.4(B:I0) IC156.7(1Y)
634354: IC18.4(B:I0) IC70.3(D1) IC155.9(2Y)
654654: IC122.8(A7) IC227.16(Q7)
4654654: IC70.1(D3) IC72.5(B:I1) IC156.9(2Y)
5434534: IC122.7(A6) IC227.15(Q6)
AD0: IC302.18(Y1)
AD7: IC302.11(Y8)
AD8: IC303.18(Y1)
AD15: IC303.11(Y8)
AD16: IC28.18(Y1)
AD17: IC28.17(Y2)
AD18: IC28.16(Y3)
AD19: IC28.15(Y4)
ADDR_ADDER_PC_OR_MAR: IC161.1(!A!/B) IC196.1(!A!/B) IC211.1(!A!/B) IC212.1(!A!/B)
ADDR_OFFSET_SRC: IC268.1(!A!/B) IC278.1(!A!/B)
ADDR_SEGMENT_SRC_0: IC273.14(A) IC274.14(A) IC275.14(A) IC276.14(A) IC279.14(A) IC280.14(A) IC281.14(A) IC282.14(A)
ADDR_SEGMENT_SRC_1: IC273.2(B) IC274.2(B) IC275.2(B) IC276.2(B) IC279.2(B) IC280.2(B) IC281.2(B) IC282.2(B)
AH_OUT: IC102.1(G1) IC102.19(G2)
AH_WRT: IC123.1(G)
AL_OUT: IC117.1(G1) IC117.19(G2)
AL_WRT: IC1.1(G)
ALU_0: IC14.9(F0) IC257.2(1A)
ALU_1: IC14.10(F1) IC257.5(2A)
ALU_2: IC14.11(F2) IC257.11(3A)
ALU_3: IC14.13(F3) IC257.14(4A)
ALU_4: IC15.9(F0) IC258.2(1A)
ALU_5: IC15.10(F1) IC258.5(2A)
ALU_6: IC15.11(F2) IC258.11(3A)
ALU_7: IC15.13(F3) IC257.3(1B) IC257.6(2B) IC257.10(3B) IC257.13(4B) IC258.3(1B) IC258.6(2B) IC258.10(3B) IC258.13(4B) IC258.14(4A)
ALU_CF_IN_SRC0: IC167.1(!A!/B)
ALU_CF_IN_SRC1: IC56.14(A)
ALU_CF_IN_SRC2: IC56.2(B)
ALU_CF_OUT_INV: IC58.1(A:I0)
ALU_FINAL_CF: IC58.3(A:O) IC126.4(2D) IC155.12(2C2) IC243.5(1C1)
ALU_MODE: IC14.8(M) IC15.8(M)
ALU_OP0: IC14.6(S0) IC15.6(S0) IC131.3(A:I1) IC138.13(A:I2)
ALU_OP1: IC14.5(S1) IC15.5(S1) IC65.2(A:I0) IC141.13(A:I2)
ALU_OP2: IC14.4(S2) IC15.4(S2) IC65.3(A:I1) IC141.1(A:I0)
ALU_OP3: IC14.3(S3) IC15.3(S3) IC131.2(A:I0) IC138.2(A:I1)
ALU_OUT_SRC: IC257.1(!A!/B) IC258.1(!A!/B)
AUX_FLAGS_OUT: IC116.1(G1) IC116.19(G2)
AUX_FLAGS_WRT: IC128.1(M) IC128.2(N) IC144.1(M) IC144.2(N)
BH_OUT: IC3.1(G1) IC3.19(G2)
BH_WRT: IC153.1(G)
BL_OUT: IC9.1(G1) IC9.19(G2)
BL_WRT: IC100.1(G)
BPH_OUT: IC114.1(G1)
BPH_WRT: IC99.1(G)
BPL_OUT: IC113.1(G1)
BPL_WRT: IC98.1(G)
CF: IC122.3(A2) IC155.10(2C0) IC167.2(1A) IC227.5(Q2) IC243.6(1C0)
CF_FROM_ALU: IC15.16(CN+4) IC58.2(A:I1)
CF_FROM_SHR_MACHINE: IC19.2(1Q) IC91.2(A1) IC243.4(1C2)
CF_IN_SRC_0: IC243.14(A)
CF_IN_SRC_1: IC243.2(B)
CH_OUT: IC146.1(G1) IC146.19(G2)
CH_WRT: IC185.1(G)
CL_OUT: IC2.1(G1) IC2.19(G2)
CL_WRT: IC101.1(G)
CLK: IC7.11(CLK) IC60.11(CLK) IC61.11(CLK) IC62.11(CLK) IC75.11(CLK) IC76.11(CLK) IC77.11(CLK) IC78.11(CLK) IC79.11(CLK) IC128.7(CLK) IC134.11(CLK) IC135.11(CLK) IC136.11(CLK) IC137.11(CLK) IC144.7(CLK) IC162.11(CLK) IC189.11(CLK) IC204.3(A:CLK) IC248.7(CLK) IC249.7(CLK) IC410.4(B:O) IC412.14(D1)
COND_0: IC70.11(A)
COND_1: IC70.10(B)
COND_2: IC70.9(C)
COND_SRC_0: IC155.14(A) IC156.14(A)
COND_SRC_1: IC155.2(B) IC156.2(B)
CONDITION: IC70.5(Y) IC74.5(B:I1)
CS_H_0: IC275.6(1C0)
CS_H_1: IC275.10(2C0)
CS_H_2: IC276.6(1C0)
CS_H_3: IC276.10(2C0)
CS_H_4: IC273.6(1C0)
CS_H_5: IC273.10(2C0)
CS_H_6: IC274.6(1C0)
CS_H_7: IC274.10(2C0)
CS_H_OUT: IC140.1(G1) IC140.19(G2)
CS_H_WRT: IC173.1(G)
CS_L_0: IC282.6(1C0)
CS_L_1: IC282.10(2C0)
CS_L_2: IC279.6(1C0)
CS_L_3: IC279.10(2C0)
CS_L_4: IC280.6(1C0)
CS_L_5: IC280.10(2C0)
CS_L_6: IC281.6(1C0)
CS_L_7: IC281.10(2C0)
CS_L_OUT: IC210.1(G1) IC210.19(G2)
CS_L_WRT: IC205.1(G)
DATA0: IC118.3(1D) IC169.3(1D) IC179.18(A:Y1) IC295.18(A:Y1)
DATA1: IC118.4(2D) IC169.4(2D) IC179.16(A:Y2) IC295.16(A:Y2)
DATA2: IC118.7(3D) IC169.7(3D) IC179.14(A:Y3) IC295.14(A:Y3)
DATA3: IC118.8(4D) IC169.8(4D) IC179.12(A:Y4) IC295.12(A:Y4)
DATA4: IC118.13(5D) IC169.13(5D) IC178.18(A:Y1) IC294.18(A:Y1)
DATA5: IC118.14(6D) IC169.14(6D) IC178.16(A:Y2) IC294.16(A:Y2)
DATA6: IC118.17(7D) IC169.17(7D) IC178.14(A:Y3) IC294.14(A:Y3)
DATA7: IC118.18(8D) IC169.18(8D) IC178.12(A:Y4) IC294.12(A:Y4)
DH_OUT: IC145.1(G1) IC145.19(G2)
DH_WRT: IC184.1(G)
DI_H_OUT: IC267.1(G1) IC267.19(G2)
DI_H_WRT: IC254.1(G)
DI_L_OUT: IC266.1(G1) IC266.19(G2)
DI_L_WRT: IC265.1(G)
DIR: IC116.8(A7) IC128.5(Q3)
DL_OUT: IC245.1(G1) IC245.19(G2)
DMA_ACK: IC116.2(A1) IC144.3(Q1)
DMA_PENDING: IC43.3(B:I) IC238.4(B:I0) IC269.3(A:O)
DMA_REQ: IC204.2(A:D) R14.2
DMA_TRISTATE: IC116.3(A2) IC144.4(Q2) IC250.4(B:I0)
DS_H_0: IC275.5(1C1)
DS_H_1: IC275.11(2C1)
DS_H_2: IC276.5(1C1)
DS_H_3: IC276.11(2C1)
DS_H_4: IC273.5(1C1)
DS_H_5: IC273.11(2C1)
DS_H_6: IC274.5(1C1)
DS_H_7: IC274.11(2C1)
DS_H_OUT: IC215.1(G1) IC215.19(G2)
DS_H_WRT: IC165.1(G)
DS_L_0: IC282.5(1C1)
DS_L_1: IC282.11(2C1)
DS_L_2: IC279.5(1C1)
DS_L_3: IC279.11(2C1)
DS_L_4: IC280.5(1C1)
DS_L_5: IC280.11(2C1)
DS_L_6: IC281.5(1C1)
DS_L_7: IC281.11(2C1)
DS_L_OUT: IC171.1(G1) IC171.19(G2)
DS_L_WRT: IC166.1(G)
ENCODED_INT_STATUS_OUT: IC154.1(G1) IC154.19(G2)
ES_H_0: IC275.3(1C3)
ES_H_1: IC275.13(2C3)
ES_H_2: IC276.3(1C3)
ES_H_3: IC276.13(2C3)
ES_H_4: IC273.3(1C3)
ES_H_5: IC273.13(2C3)
ES_H_6: IC274.3(1C3)
ES_H_7: IC274.13(2C3)
ES_H_OUT: IC264.1(G1) IC264.19(G2)
ES_H_WRT: IC261.1(G)
ES_L_0: IC282.3(1C3)
ES_L_1: IC282.13(2C3)
ES_L_2: IC279.3(1C3)
ES_L_3: IC279.13(2C3)
ES_L_4: IC280.3(1C3)
ES_L_5: IC280.13(2C3)
ES_L_6: IC281.3(1C3)
ES_L_7: IC281.13(2C3)
ES_L_OUT: IC263.1(G1) IC263.19(G2)
ES_L_WRT: IC262.1(G)
FINAL_CONDITION: IC74.6(B:O) IC83.3(B:I)
FINAL_MEM_IO: IC69.5(B:Y3) RN4.14
FINAL_RD: IC69.9(B:Y1) RN4.16
FINAL_WR: IC69.7(B:Y2) RN4.15
FLAGS_REG_OUT: IC122.1(G1) IC122.19(G2)
GND: IC22.15(G) IC23.15(G) IC49.5(2A) IC49.11(3A) IC49.14(4A) IC49.15(G) IC50.7(C0) IC55.2(1A) IC55.5(2A) IC55.11(3A) IC55.14(4A) IC55.15(G) IC56.1(1G) IC56.6(1C0) IC56.15(2G) IC63.2(1A) IC63.5(2A) IC63.11(3A) IC63.14(4A) IC63.15(G) IC68.2(1A) IC68.5(2A) IC68.11(3A) IC68.14(4A) IC68.15(G) IC69.17(B:A4) IC70.7(G) IC86.15(G) IC88.15(G) IC89.15(G) IC90.15(G) IC95.7(C0) IC115.2(A1) IC115.3(A2) IC115.4(A3) IC115.5(A4) IC115.6(A5) IC115.7(A6) IC115.8(A7) IC115.9(A8) IC121.15(G) IC128.9(G1) IC128.10(G2) IC142.3(D1) IC144.9(G1) IC144.10(G2) IC154.2(A1) IC154.3(A2) IC154.4(A3) IC154.8(A7) IC154.9(A8) IC155.1(1G) IC155.15(2G) IC156.1(1G) IC156.15(2G) IC159.3(D1) IC160.3(D1) IC167.15(G) IC186.3(D1) IC199.13(A:I4) IC208.4(1C2) IC226.5(EI) IC227.14(D6) IC227.17(D7) IC227.18(D8) IC248.9(G1) IC248.10(G2) IC249.9(G1) IC249.10(G2) IC255.4(1C2) IC256.4(1C2) IC258.15(G) IC285.3(A2) IC285.5(A1) IC285.7(C0) IC285.12(A4) IC285.14(A3) IC287.2(B2) IC287.6(B1) IC287.11(B4) IC287.15(B3) IC412.9(G1) IC412.10(G2) R1.1 R5.1 R6.1 R7.1 R8.1 R10.1 R11.1 R12.1 R13.1 R14.1 RN1.9 RN1.10 RN1.11 RN1.12 RN1.13 RN1.14 RN1.15 RN1.16 RN2.9 RN2.10 RN2.11 RN2.12 RN2.13 RN2.14 RN2.15 RN2.16 RN3.9 RN3.10 RN3.11 RN3.12 RN3.13 RN3.14 RN3.15 RN3.16 S3.2(P) S5.3(S) S6.3(S) U$1.1(A14) U$1.14(GND) U$1.20(/CE) U$1.22(/OE) U$1.27(/WE) U$2.1(A14) U$2.14(GND) U$2.20(/CE) U$2.22(/OE) U$2.27(/WE) U$3.1(A14) U$3.14(GND) U$3.20(/CE) U$3.22(/OE) U$3.27(/WE) U$4.1(A14) U$4.14(GND) U$4.20(/CE) U$4.22(/OE) U$4.27(/WE) U$5.1(A14) U$5.14(GND) U$5.20(/CE) U$5.22(/OE) U$5.27(/WE) U$6.1(A14) U$6.14(GND) U$6.20(/CE) U$6.22(/OE) U$6.27(/WE) U$7.1(A14) U$7.14(GND) U$7.20(/CE) U$7.22(/OE) U$7.27(/WE) U$8.1(A14) U$8.14(GND) U$8.20(/CE) U$8.22(/OE) U$8.27(/WE) U$9.1(A14) U$9.14(GND) U$9.20(/CE) U$9.22(/OE) U$9.27(/WE)
HALT: IC116.7(A6) IC128.4(Q2) IC415.5(B:I1)
IMM_X_OUT: IC115.1(G1) IC115.19(G2)
IMMY_OUT: IC16.1(G1) IC16.19(G2)
IN_TRAP: IC116.6(A5) IC128.3(Q1) IC270.3(B:I) IC271.3(B:I)
INT_ACK: IC222.4(G2A) IC222.5(G2B)
INT_ENABLE: IC64.2(A:I1) IC93.2(A:I1) IC116.4(A3) IC132.2(A:I1) IC144.5(Q3) IC150.2(A:I1) IC151.2(A:I1) IC157.2(A:I1) IC158.2(A:I1) IC191.2(A:I1)
INT_PENDING: IC45.2(A:I1) IC141.6(B:O) IC141.9(C:I0)
INT_REQ_0: IC8.3(A:CLK) R5.2
INT_REQ_1: IC163.3(A:CLK) R6.2
INT_REQ_2: IC164.3(A:CLK) R7.2
INT_REQ_3: IC168.3(A:CLK) R8.2
INT_REQ_4: IC174.3(A:CLK) R10.2
INT_REQ_5: IC188.3(A:CLK) R11.2
INT_REQ_6: IC221.3(A:CLK) R12.2
INT_REQ_7: IC187.3(A:CLK) R13.2
INTERRUPT_STATUS_OUT: IC125.1(G1) IC125.19(G2)
IR_0: IC129.3(D1) IC169.2(1Q)
IR_1: IC73.3(D1) IC169.5(2Q)
IR_2: IC34.3(D1) IC169.6(3Q)
IR_3: IC35.3(D1) IC169.9(4Q)
IR_4: IC36.3(D1) IC169.12(5Q)
IR_5: IC37.3(D1) IC169.15(6Q)
IR_6: IC38.3(D1) IC169.16(7Q)
IR_7: IC40.3(D1) IC169.19(8Q)
IR_8: IC41.3(D1) IC118.2(1Q)
IR_9: IC71.3(D1) IC118.5(2Q)
IR_10: IC20.3(D1) IC118.6(3Q)
IR_11: IC118.9(4Q) IC172.3(D1)
IR_H_WRT: IC118.1(G)
IR_L_WRT: IC169.1(G)
MAR_H_0: IC211.3(1B) IC277.2(1A)
MAR_H_1: IC211.6(2B) IC277.5(2A)
MAR_H_2: IC211.10(3B) IC277.11(3A)
MAR_H_3: IC211.13(4B) IC277.14(4A)
MAR_H_4: IC212.3(1B) IC278.2(1A)
MAR_H_5: IC212.6(2B) IC278.5(2A)
MAR_H_6: IC212.10(3B) IC278.11(3A)
MAR_H_7: IC212.13(4B) IC278.14(4A)
MAR_L_0: IC161.3(1B) IC268.2(1A)
MAR_L_1: IC161.6(2B) IC268.5(2A)
MAR_L_2: IC161.10(3B) IC268.11(3A)
MAR_L_3: IC161.13(4B) IC268.14(4A)
MAR_L_4: IC196.3(1B) IC272.2(1A)
MAR_L_5: IC196.6(2B) IC272.5(2A)
MAR_L_6: IC196.10(3B) IC272.11(3A)
MAR_L_7: IC196.13(4B) IC272.14(4A)
MARH_WRT: IC7.1(G)
MARH_X_OUT: IC24.19(B:G) IC25.19(B:G)
MARL_0: IC27.11(B:A1) IC189.2(1Q)
MARL_1: IC27.13(B:A2) IC189.5(2Q)
MARL_WRT: IC189.1(G)
MARL_X_OUT: IC26.19(B:G) IC27.19(B:G)
MASK_0: IC82.9(C:I0) IC244.11(B:A1) IC248.3(Q1)
MASK_1: IC152.9(C:I0) IC244.13(B:A2) IC248.4(Q2)
MASK_2: IC201.9(C:I0) IC244.15(B:A3) IC248.5(Q3)
MASK_3: IC203.9(C:I0) IC244.17(B:A4) IC248.6(Q4)
MASK_4: IC206.9(C:I0) IC247.11(B:A1) IC249.3(Q1)
MASK_5: IC228.9(C:I0) IC247.13(B:A2) IC249.4(Q2)
MASK_6: IC190.9(C:I0) IC247.15(B:A3) IC249.5(Q3)
MASK_7: IC242.9(C:I0) IC247.17(B:A4) IC249.6(Q4)
MASK_ENABLE: IC82.10(C:I1) IC116.5(A4) IC144.6(Q4) IC152.10(C:I1) IC190.10(C:I1) IC201.10(C:I1) IC203.10(C:I1) IC206.10(C:I1) IC228.10(C:I1) IC242.10(C:I1)
MASK_FLAGS_OUT: IC244.19(B:G) IC247.19(B:G)
MASK_FLAGS_WRT: IC248.1(M) IC248.2(N) IC249.1(M) IC249.2(N)
MDR_IN_BUS0: IC21.3(1D) IC180.3(1D)
MDR_IN_BUS1: IC21.4(2D) IC180.4(2D)
MDR_IN_BUS2: IC21.7(3D) IC180.7(3D)
MDR_IN_BUS3: IC21.8(4D) IC180.8(4D)
MDR_IN_BUS4: IC21.13(5D) IC180.13(5D)
MDR_IN_BUS5: IC21.14(6D) IC180.14(6D)
MDR_IN_BUS6: IC21.17(7D) IC180.17(7D)
MDR_IN_BUS7: IC21.18(8D) IC180.18(8D)
MDR_IN_BUS8: IC296.3(1D) IC301.3(1D)
MDR_IN_BUS9: IC296.4(2D) IC301.4(2D)
MDR_IN_BUS10: IC296.7(3D) IC301.7(3D)
MDR_IN_BUS11: IC296.8(4D) IC301.8(4D)
MDR_IN_BUS12: IC296.13(5D) IC301.13(5D)
MDR_IN_BUS13: IC296.14(6D) IC301.14(6D)
MDR_IN_BUS14: IC296.17(7D) IC301.17(7D)
MDR_IN_BUS15: IC296.18(8D) IC301.18(8D)
MDR_IN_SRC: IC22.1(!A!/B) IC23.1(!A!/B)
MDRH_H_DATA_OUT: IC294.1(A:G) IC295.1(A:G)
MDRH_H_WRT: IC296.1(G)
MDRH_H_X_OUT: IC297.1(A:G) IC298.1(A:G)
MDRH_H_Y_OUT: IC299.1(A:G) IC300.1(A:G)
MDRH_L_DATA_OUT: IC292.1(A:G) IC293.1(A:G)
MDRH_L_WRT: IC301.1(G)
MDRH_L_X_OUT: IC290.1(A:G) IC291.1(A:G)
MDRH_L_Y_OUT: IC288.1(A:G) IC289.1(A:G)
MDRL_H_DATA_OUT: IC178.1(A:G) IC179.1(A:G)
MDRL_H_WRT: IC180.1(G)
MDRL_H_X_OUT: IC176.1(A:G) IC181.1(A:G)
MDRL_H_Y_OUT: IC182.1(A:G) IC183.1(A:G)
MDRL_L_DATA_OUT: IC30.1(A:G) IC31.1(A:G)
MDRL_L_WRT: IC21.1(G)
MDRL_L_X_OUT: IC12.1(A:G) IC13.1(A:G)
MDRL_L_Y_OUT: IC10.1(A:G) IC11.1(A:G)
MEM_IO: IC60.6(Q3) IC69.15(B:A3)
MUX_A: IC213.3(A:O)
MUX_B: IC235.8(C:O)
MUX_C: IC236.8(C:O)
N$1: IC1.2(1Q) IC117.2(A1)
N$2: IC1.5(2Q) IC117.3(A2)
N$3: IC1.6(3Q) IC117.4(A3)
N$4: IC1.9(4Q) IC117.5(A4)
N$5: IC1.12(5Q) IC117.6(A5)
N$6: IC1.15(6Q) IC117.7(A6)
N$7: IC102.8(A7) IC123.16(7Q)
N$8: IC1.19(8Q) IC117.9(A8)
N$9: IC29.6(A5) IC44.6(A5) IC544.12(5Q)
N$10: IC80.6(B:O) IC133.2(A:I1)
N$11: IC46.3(A:O) IC155.3(1C3)
N$12: IC49.4(1Y) IC50.6(B1)
N$13: IC9.2(A1) IC100.2(1Q)
N$14: IC49.7(2Y) IC50.2(B2)
N$15: IC9.3(A2) IC100.5(2Q)
N$16: IC9.4(A3) IC100.6(3Q)
N$17: IC9.5(A4) IC100.9(4Q)
N$18: IC9.6(A5) IC100.12(5Q)
N$19: IC9.7(A6) IC100.15(6Q)
N$20: IC9.8(A7) IC100.16(7Q)
N$21: IC9.9(A8) IC100.19(8Q)
N$22: IC56.3(1C3) IC57.2(A:O)
N$23: IC65.1(A:O) IC138.1(A:I0)
N$24: IC143.3(A:O) IC170.5(B:I1)
N$25: IC2.2(A1) IC101.2(1Q)
N$26: IC2.3(A2) IC101.5(2Q)
N$27: IC2.4(A3) IC101.6(3Q)
N$28: IC2.5(A4) IC101.9(4Q)
N$29: IC2.6(A5) IC101.12(5Q)
N$30: IC2.7(A6) IC101.15(6Q)
N$31: IC2.8(A7) IC101.16(7Q)
N$32: IC2.9(A8) IC101.19(8Q)
N$33: IC56.4(1C2) IC57.1(A:I) IC167.4(1Y)
N$34: IC131.1(A:O) IC141.2(A:I1)
N$35: IC49.9(3Y) IC50.15(B3)
N$36: IC49.12(4Y) IC50.11(B4)
N$37: IC51.6(B1) IC55.4(1Y)
N$38: IC51.2(B2) IC55.7(2Y)
N$39: IC51.15(B3) IC55.9(3Y)
N$40: IC51.11(B4) IC55.12(4Y)
N$41: IC227.3(D1) IC241.7(1Y)
N$42: IC179.2(A:A1) IC180.2(1Q) IC181.2(A:A1) IC182.2(A:A1)
N$43: IC179.4(A:A2) IC180.5(2Q) IC181.4(A:A2) IC182.4(A:A2)
N$44: IC179.6(A:A3) IC180.6(3Q) IC181.6(A:A3) IC182.6(A:A3)
N$45: IC179.8(A:A4) IC180.9(4Q) IC181.8(A:A4) IC182.8(A:A4)
N$46: IC176.2(A:A1) IC178.2(A:A1) IC180.12(5Q) IC183.2(A:A1)
N$47: IC176.4(A:A2) IC178.4(A:A2) IC180.15(6Q) IC183.4(A:A2)
N$48: IC176.6(A:A3) IC178.6(A:A3) IC180.16(7Q) IC183.6(A:A3)
N$49: IC204.5(A:Q) IC269.1(A:I0)
N$50: IC66.2(A:I0) IC130.6(B:O) IC143.2(A:I1)
N$51: IC176.8(A:A4) IC178.8(A:A4) IC180.19(8Q) IC183.8(A:A4)
N$52: IC27.15(B:A3) IC189.6(3Q)
N$53: IC27.17(B:A4) IC189.9(4Q)
N$54: IC26.11(B:A1) IC189.12(5Q)
N$55: IC26.13(B:A2) IC189.15(6Q)
N$56: IC26.15(B:A3) IC189.16(7Q)
N$57: IC26.17(B:A4) IC189.19(8Q)
N$58: IC7.2(1Q) IC25.11(B:A1)
N$59: IC7.5(2Q) IC25.13(B:A2)
N$60: IC7.6(3Q) IC25.15(B:A3)
N$61: IC7.9(4Q) IC25.17(B:A4)
N$62: IC7.12(5Q) IC24.11(B:A1)
N$63: IC7.15(6Q) IC24.13(B:A2)
N$64: IC7.16(7Q) IC24.15(B:A3)
N$65: IC52.6(B1) IC63.4(1Y)
N$66: IC122.9(A8) IC227.19(Q8)
N$67: IC5.2(1Q) IC109.11(B:A1)
N$68: IC5.5(2Q) IC109.13(B:A2)
N$69: IC5.6(3Q) IC109.15(B:A3)
N$70: IC5.9(4Q) IC109.17(B:A4)
N$71: IC5.12(5Q) IC110.11(B:A1)
N$72: IC5.15(6Q) IC110.13(B:A2)
N$73: IC7.19(8Q) IC24.17(B:A4)
N$74: IC52.2(B2) IC63.7(2Y)
N$75: IC52.15(B3) IC63.9(3Y)
N$76: IC54.2(1Q) IC87.2(A1) IC139.2(A1)
N$77: IC75.3(D1) U$1.11(I/O0)
N$78: IC42.2(A:I1) IC94.4(B:O)
N$79: IC32.3(D1) IC186.5(Y)
N$80: IC83.4(B:O) IC85.13(A:I2)
N$81: IC53.15(B3) IC68.9(3Y)
N$82: IC66.1(A:O) IC170.4(B:I0)
N$83: IC10.2(A:A1) IC13.2(A:A1) IC21.2(1Q) IC30.2(A:A1)
N$84: IC133.1(A:I0) IC170.6(B:O)
N$85: IC66.3(A:I1) IC138.12(A:O)
N$86: IC59.1(A:I) IC209.6(B:O)
N$87: IC145.2(A1) IC184.2(1Q)
N$88: IC227.4(D2) IC243.7(1Y)
N$89: IC141.12(A:O) IC143.1(A:I0)
N$90: IC227.7(D3) IC255.7(1Y)
N$91: IC53.11(B4) IC68.12(4Y)
N$92: IC227.8(D4) IC256.7(1Y)
N$93: IC208.7(1Y) IC227.13(D5)
N$94: IC213.1(A:I0) IC214.6(B:O)
N$95: IC39.1(A:CLR) IC42.3(A:O)
N$96: IC121.4(1Y) IC126.3(1D)
N$97: IC32.4(D2) IC160.5(Y)
N$98: IC257.4(1Y) RN5.16
N$99: IC257.7(2Y) RN5.15
N$100: IC257.9(3Y) RN5.14
N$101: IC257.12(4Y) RN5.13
N$102: IC258.4(1Y) RN5.12
N$103: IC258.7(2Y) RN5.11
N$104: IC258.9(3Y) RN5.10
N$105: IC258.12(4Y) RN5.9
N$106: IC99.19(8Q) IC114.9(A8)
N$107: IC14.16(CN+4) IC15.7(CN)
N$108: IC39.5(A:Q) IC47.2(A:I1)
N$109: IC145.3(A2) IC184.5(2Q)
N$110: IC1.16(7Q) IC117.8(A7)
N$111: IC145.4(A3) IC184.6(3Q)
N$112: IC145.5(A4) IC184.9(4Q)
N$113: IC32.7(D3) IC159.5(Y)
N$114: IC19.3(1D) IC89.4(1Y)
N$115: IC19.4(2D) IC89.7(2Y)
N$116: IC19.7(3D) IC89.9(3Y)
N$117: IC19.8(4D) IC89.12(4Y)
N$118: IC19.13(5D) IC86.4(1Y)
N$119: IC19.14(6D) IC86.7(2Y)
N$120: IC19.17(7D) IC86.9(3Y)
N$121: IC19.18(8D) IC86.12(4Y)
N$122: IC17.3(1D) IC90.4(1Y)
N$123: IC17.4(2D) IC90.7(2Y)
N$124: IC17.7(3D) IC90.9(3Y)
N$125: IC17.8(4D) IC90.12(4Y)
N$126: IC17.13(5D) IC88.4(1Y)
N$127: IC17.14(6D) IC88.7(2Y)
N$128: IC17.17(7D) IC88.9(3Y)
N$129: IC17.18(8D) IC88.12(4Y)
N$130: IC214.4(B:I0) IC229.3(A:O)
N$131: IC93.13(A:I2) IC125.2(A1) IC162.2(Q1)
N$132: IC10.4(A:A2) IC13.4(A:A2) IC21.5(2Q) IC30.4(A:A2)
N$133: IC82.8(C:O) IC93.1(A:I0)
N$134: IC10.6(A:A3) IC13.6(A:A3) IC21.6(3Q) IC30.6(A:A3)
N$135: IC145.6(A5) IC184.12(5Q)
N$136: IC145.7(A6) IC184.15(6Q)
N$137: IC10.8(A:A4) IC13.8(A:A4) IC21.9(4Q) IC30.8(A:A4)
N$138: IC11.2(A:A1) IC12.2(A:A1) IC21.12(5Q) IC31.2(A:A1)
N$139: IC145.8(A7) IC184.16(7Q)
N$140: IC11.4(A:A2) IC12.4(A:A2) IC21.15(6Q) IC31.4(A:A2)
N$141: IC11.6(A:A3) IC12.6(A:A3) IC21.16(7Q) IC31.6(A:A3)
N$142: IC145.9(A8) IC184.19(8Q)
N$143: IC5.16(7Q) IC110.15(B:A3)
N$144: IC52.11(B4) IC63.12(4Y)
N$145: IC53.6(B1) IC68.4(1Y)
N$146: IC5.19(8Q) IC110.17(B:A4)
N$147: IC53.2(B2) IC68.7(2Y)
N$148: IC48.7(3D) IC96.9(3Y)
N$149: IC48.8(4D) IC96.12(4Y)
N$150: IC95.5(A1) IC161.4(1Y)
N$151: IC4.2(1Q) IC111.11(B:A1)
N$152: IC49.1(!A!/B) IC55.1(!A!/B) IC63.1(!A!/B) IC68.1(!A!/B) IC85.12(A:O)
N$153: IC32.8(D4) IC142.5(Y)
N$154: IC84.4(B:O) IC85.2(A:I1)
N$155: IC268.15(G) IC272.15(G) IC277.15(G) IC278.15(G)
N$156: IC48.13(5D) IC97.4(1Y)
N$157: IC48.14(6D) IC97.7(2Y)
N$158: IC48.17(7D) IC97.9(3Y)
N$159: IC48.18(8D) IC97.12(4Y)
N$160: IC6.3(1D) IC103.4(1Y)
N$161: IC6.4(2D) IC103.7(2Y)
N$162: IC6.7(3D) IC103.9(3Y)
N$163: IC6.8(4D) IC103.12(4Y)
N$164: IC11.8(A:A4) IC12.8(A:A4) IC21.19(8Q) IC31.8(A:A4)
N$165: IC6.13(5D) IC104.4(1Y)
N$166: IC6.14(6D) IC104.7(2Y)
N$167: IC54.5(2Q) IC87.3(A2) IC139.3(A2)
N$168: IC6.17(7D) IC104.9(3Y)
N$169: IC10.18(A:Y1)
N$170: IC10.16(A:Y2)
N$171: IC10.14(A:Y3)
N$172: IC10.12(A:Y4)
N$173: IC229.2(A:I1) IC230.4(B:O) IC235.10(C:I1) IC237.2(A:I1)
N$174: IC32.13(D5) IC129.5(Y)
N$175: IC32.14(D6) IC73.5(Y)
N$176: IC14.7(CN) IC56.7(1Y)
N$177: IC13.18(A:Y1)
N$178: IC13.16(A:Y2)
N$179: IC13.14(A:Y3)
N$180: IC13.12(A:Y4)
N$181: IC12.18(A:Y1)
N$182: IC12.16(A:Y2)
N$183: IC12.14(A:Y3)
N$184: IC12.12(A:Y4)
N$185: IC32.17(D7) IC34.5(Y)
N$186: IC32.18(D8) IC35.5(Y)
N$187: IC33.3(D1) IC36.5(Y)
N$188: IC33.4(D2) IC37.5(Y)
N$189: IC33.7(D3) IC38.5(Y)
N$190: IC33.8(D4) IC40.5(Y)
N$191: IC22.7(2Y)
N$192: IC22.9(3Y)
N$193: IC22.12(4Y)
N$194: IC23.4(1Y)
N$195: IC23.7(2Y)
N$196: IC23.9(3Y)
N$197: IC23.12(4Y)
N$198: IC22.3(1B)
N$199: IC22.6(2B)
N$200: IC30.18(A:Y1)
N$201: IC30.16(A:Y2)
N$202: IC95.4(S1) IC96.2(1A)
N$203: IC30.14(A:Y3)
N$204: IC30.12(A:Y4)
N$205: IC95.1(S2) IC96.5(2A)
N$206: IC31.18(A:Y1)
N$207: IC31.16(A:Y2)
N$208: IC31.14(A:Y3)
N$209: IC31.12(A:Y4)
N$210: IC22.4(1Y)
N$211: IC22.10(3B)
N$212: IC22.13(4B)
N$213: IC23.3(1B)
N$214: IC23.6(2B)
N$215: IC23.10(3B)
N$216: IC23.13(4B)
N$217: IC116.9(A8) IC128.6(Q4)
N$218: IC33.13(D5) IC41.5(Y)
N$219: IC33.14(D6) IC71.5(Y)
N$220: IC8.5(A:Q) IC162.3(D1)
N$221: IC102.6(A5) IC123.12(5Q)
N$222: IC195.2(A:I1) IC222.15(Y0)
N$223: IC8.1(A:CLR) IC195.3(A:O)
N$224: IC95.13(S3) IC96.11(3A)
N$225: IC20.5(Y) IC33.17(D7)
N$226: IC93.12(A:O) IC226.4
N$227: IC95.10(S4) IC96.14(4A)
N$228: IC33.18(D8) IC172.5(Y)
N$229: IC102.7(A6) IC123.15(6Q)
N$230: IC205.2(1Q) IC210.2(A1)
N$231: IC120.3(A:O) IC241.4(1C2)
N$232: IC97.2(1A) IC119.4(S1)
N$233: IC97.5(2A) IC119.1(S2)
N$234: IC205.5(2Q) IC210.3(A2)
N$235: IC102.9(A8) IC123.19(8Q)
N$236: IC102.2(A1) IC123.2(1Q)
N$237: IC102.3(A2) IC123.5(2Q)
N$238: IC102.4(A3) IC123.6(3Q)
N$239: IC205.6(3Q) IC210.4(A3)
N$240: IC205.9(4Q) IC210.5(A4)
N$241: IC205.12(5Q) IC210.6(A5)
N$242: IC205.15(6Q) IC210.7(A6)
N$243: IC205.16(7Q) IC210.8(A7)
N$244: IC205.19(8Q) IC210.9(A8)
N$245: IC140.2(A1) IC173.2(1Q)
N$246: IC140.3(A2) IC173.5(2Q)
N$247: IC140.4(A3) IC173.6(3Q)
N$248: IC140.5(A4) IC173.9(4Q)
N$249: IC102.5(A4) IC123.9(4Q)
N$250: IC140.6(A5) IC173.12(5Q)
N$251: U$2.10(A0)
N$252: U$2.9(A1)
N$253: U$2.8(A2)
N$254: U$2.7(A3)
N$255: U$2.6(A4)
N$256: U$2.5(A5)
N$257: U$2.4(A6)
N$258: U$2.3(A7)
N$259: U$2.25(A8)
N$260: U$2.24(A9)
N$261: U$2.21(A10)
N$262: U$2.23(A11)
N$263: U$2.2(A12)
N$264: U$2.26(A13)
N$265: U$3.10(A0)
N$266: U$3.9(A1)
N$267: U$3.8(A2)
N$268: U$3.7(A3)
N$269: U$3.6(A4)
N$270: U$3.5(A5)
N$271: U$3.4(A6)
N$272: U$3.3(A7)
N$273: U$3.25(A8)
N$274: U$3.24(A9)
N$275: U$3.21(A10)
N$276: U$3.23(A11)
N$277: U$3.2(A12)
N$278: U$3.26(A13)
N$279: U$4.10(A0)
N$280: U$4.9(A1)
N$281: U$4.8(A2)
N$282: U$4.7(A3)
N$283: U$4.6(A4)
N$284: U$4.5(A5)
N$285: U$4.4(A6)
N$286: U$4.3(A7)
N$287: U$4.25(A8)
N$288: U$4.24(A9)
N$289: U$4.21(A10)
N$290: U$4.23(A11)
N$291: U$4.2(A12)
N$292: U$4.26(A13)
N$293: U$5.10(A0)
N$294: U$5.9(A1)
N$295: U$5.8(A2)
N$296: U$5.7(A3)
N$297: U$5.6(A4)
N$298: U$5.5(A5)
N$299: U$5.4(A6)
N$300: U$5.3(A7)
N$301: U$5.25(A8)
N$302: U$5.24(A9)
N$303: U$5.21(A10)
N$304: U$5.23(A11)
N$305: U$5.2(A12)
N$306: U$5.26(A13)
N$307: IC140.7(A6) IC173.15(6Q)
N$308: IC140.8(A7) IC173.16(7Q)
N$309: IC140.9(A8) IC173.19(8Q)
N$310: IC166.2(1Q) IC171.2(A1)
N$311: IC166.5(2Q) IC171.3(A2)
N$312: IC97.11(3A) IC119.13(S3)
N$313: IC97.14(4A) IC119.10(S4)
N$314: IC103.2(1A) IC124.4(S1)
N$315: IC166.6(3Q) IC171.4(A3)
N$316: IC103.5(2A) IC124.1(S2)
N$317: IC103.11(3A) IC124.13(S3)
N$318: IC103.14(4A) IC124.10(S4)
N$319: IC104.2(1A) IC148.4(S1)
N$320: IC154.7(A6) IC226.9(A0)
N$321: IC104.5(2A) IC148.1(S2)
N$322: IC175.6(B:O) IC177.4(B:I0)
N$323: IC104.11(3A) IC148.13(S3)
N$324: IC177.6(B:O) IC192.4(B:I0)
N$325: IC3.2(A1) IC153.2(1Q)
N$326: IC3.3(A2) IC153.5(2Q)
N$327: IC3.4(A3) IC153.6(3Q)
N$328: IC3.5(A4) IC153.9(4Q)
N$329: IC3.6(A5) IC153.12(5Q)
N$330: IC3.7(A6) IC153.15(6Q)
N$331: IC3.8(A7) IC153.16(7Q)
N$332: IC3.9(A8) IC153.19(8Q)
N$333: IC50.5(A1)
N$334: IC50.3(A2)
N$335: IC50.14(A3)
N$336: IC50.12(A4)
N$337: IC52.5(A1)
N$338: IC51.5(A1)
N$339: IC51.3(A2)
N$340: IC51.14(A3)
N$341: IC51.12(A4)
N$342: IC146.2(A1) IC185.2(1Q)
N$343: IC104.14(4A) IC148.10(S4)
N$344: IC166.9(4Q) IC171.5(A4)
N$345: IC166.12(5Q) IC171.6(A5)
N$346: IC158.1(A:I0) IC190.8(C:O)
N$347: IC121.3(1B) IC127.3(A:O)
N$348: IC119.9(C4) IC124.7(C0)
N$349: IC149.3(B:I) IC226.14(GS)
N$350: IC52.3(A2)
N$351: IC52.14(A3)
N$352: IC52.12(A4)
N$353: IC53.5(A1)
N$354: IC53.3(A2)
N$355: IC158.12(A:O) IC226.11
N$356: IC141.4(B:I1) IC149.4(B:O)
N$357: IC50.9(C4) IC51.7(C0)
N$358: IC51.9(C4) IC52.7(C0)
N$359: IC52.9(C4) IC53.7(C0)
N$360: IC76.5(Q2)
N$361: IC141.3(B:I0) IC226.15(EO)
N$362: IC192.6(B:O) IC193.4(B:I0)
N$363: IC166.15(6Q) IC171.7(A6)
N$364: IC76.6(Q3)
N$365: IC64.12(A:O) IC226.3
N$366: IC64.13(A:I2) IC125.3(A2) IC162.5(Q2)
N$367: IC75.4(D2) U$1.12(I/O1)
N$368: IC132.1(A:I0) IC201.8(C:O)
N$369: IC75.7(D3) U$1.13(I/O2)
N$370: IC166.16(7Q) IC171.8(A7)
N$371: IC166.19(8Q) IC171.9(A8)
N$372: IC168.1(A:CLR) IC220.3(A:O)
N$373: IC146.3(A2) IC185.5(2Q)
N$374: IC174.1(A:CLR) IC223.3(A:O)
N$375: IC75.8(D4) U$1.15(I/O3)
N$376: IC75.13(D5) U$1.16(I/O4)
N$377: IC75.14(D6) U$1.17(I/O5)
N$378: IC60.3(D1) U$10.11(I/O0)
N$379: IC60.4(D2) U$10.12(I/O1)
N$380: IC60.7(D3) U$10.13(I/O2)
N$381: IC60.8(D4) U$10.15(I/O3)
N$382: IC60.13(D5) U$10.16(I/O4)
N$383: IC60.14(D6) U$10.17(I/O5)
N$384: IC60.17(D7) U$10.18(I/O6)
N$385: IC60.18(D8) U$10.19(I/O7)
N$386: IC61.3(D1) U$11.11(I/O0)
N$387: IC61.4(D2) U$11.12(I/O1)
N$388: IC188.1(A:CLR) IC224.3(A:O)
N$389: IC162.18(D8) IC187.5(A:Q)
N$390: IC162.4(D2) IC163.5(A:Q)
N$391: IC76.9(Q4)
N$392: IC162.7(D3) IC164.5(A:Q)
N$393: IC162.8(D4) IC168.5(A:Q)
N$394: IC162.13(D5) IC174.5(A:Q)
N$395: IC162.14(D6) IC188.5(A:Q)
N$396: IC162.17(D7) IC221.5(A:Q)
N$397: IC207.1(A:I0) IC222.7(Y7)
N$398: IC218.2(A:I1) IC222.14(Y1)
N$399: IC219.2(A:I1) IC222.13(Y2)
N$400: IC76.12(Q5)
N$401: IC76.15(Q6)
N$402: IC76.16(Q7)
N$403: IC222.11(Y4) IC223.1(A:I0)
N$404: IC4.5(2Q) IC111.13(B:A2)
N$405: IC222.9(Y6) IC225.1(A:I0)
N$406: IC187.1(A:CLR) IC207.3(A:O)
N$407: IC251.2(1Q) IC252.2(A1)
N$408: IC163.1(A:CLR) IC218.3(A:O)
N$409: IC164.1(A:CLR) IC219.3(A:O)
N$410: IC221.1(A:CLR) IC225.3(A:O)
N$411: IC125.4(A3) IC132.13(A:I2) IC162.6(Q3)
N$412: IC125.5(A4) IC150.13(A:I2) IC162.9(Q4)
N$413: IC132.12(A:O) IC226.2
N$414: IC125.6(A5) IC151.13(A:I2) IC162.12(Q5)
N$415: IC150.1(A:I0) IC203.8(C:O)
N$416: IC150.12(A:O) IC226.1
N$417: IC151.1(A:I0) IC206.8(C:O)
N$418: IC151.12(A:O) IC226.13
N$419: IC157.1(A:I0) IC228.8(C:O)
N$420: IC157.12(A:O) IC226.12
N$421: IC191.1(A:I0) IC242.8(C:O)
N$422: IC146.4(A3) IC185.6(3Q)
N$423: IC146.5(A4) IC185.9(4Q)
N$424: IC146.6(A5) IC185.12(5Q)
N$425: IC146.7(A6) IC185.15(6Q)
N$426: IC146.8(A7) IC185.16(7Q)
N$427: IC146.9(A8) IC185.19(8Q)
N$428: IC216.2(1Q) IC245.2(A1)
N$429: IC216.5(2Q) IC245.3(A2)
N$430: IC216.6(3Q) IC245.4(A3)
N$431: IC216.9(4Q) IC245.5(A4)
N$432: IC216.12(5Q) IC245.6(A5)
N$433: IC216.15(6Q) IC245.7(A6)
N$434: IC216.16(7Q) IC245.8(A7)
N$435: IC216.19(8Q) IC245.9(A8)
N$436: IC191.12(A:O) IC226.10
N$437: IC125.7(A6) IC157.13(A:I2) IC162.15(Q6)
N$438: IC125.8(A7) IC158.13(A:I2) IC162.16(Q7)
N$439: IC125.9(A8) IC162.19(Q8) IC191.13(A:I2)
N$440: IC76.19(Q8)
N$441: IC165.2(1Q) IC215.2(A1)
N$442: IC76.3(D1) U$2.11(I/O0)
N$443: IC76.4(D2) U$2.12(I/O1)
N$445: IC193.6(B:O) IC194.4(B:I0)
N$446: IC197.5(A:O) IC198.1(A:I)
N$447: IC77.5(Q2)
N$448: IC61.7(D3) U$11.13(I/O2)
N$449: IC75.17(D7) U$1.18(I/O6)
N$450: IC75.18(D8) U$1.19(I/O7)
N$451: IC76.7(D3) U$2.13(I/O2)
N$452: IC76.8(D4) U$2.15(I/O3)
N$453: IC76.13(D5) U$2.16(I/O4)
N$454: IC76.14(D6) U$2.17(I/O5)
N$455: IC76.17(D7) U$2.18(I/O6)
N$456: IC76.18(D8) U$2.19(I/O7)
N$457: IC77.3(D1) U$3.11(I/O0)
N$458: IC77.4(D2) U$3.12(I/O1)
N$459: IC77.7(D3) U$3.13(I/O2)
N$460: IC77.8(D4) U$3.15(I/O3)
N$461: IC77.13(D5) U$3.16(I/O4)
N$462: IC77.14(D6) U$3.17(I/O5)
N$463: IC77.17(D7) U$3.18(I/O6)
N$464: IC77.18(D8) U$3.19(I/O7)
N$465: IC78.3(D1) U$4.11(I/O0)
N$466: IC78.4(D2) U$4.12(I/O1)
N$467: IC78.7(D3) U$4.13(I/O2)
N$468: IC78.8(D4) U$4.15(I/O3)
N$469: IC78.13(D5) U$4.16(I/O4)
N$470: IC78.14(D6) U$4.17(I/O5)
N$471: IC78.17(D7) U$4.18(I/O6)
N$472: IC78.18(D8) U$4.19(I/O7)
N$473: IC79.3(D1) U$5.11(I/O0)
N$474: IC79.4(D2) U$5.12(I/O1)
N$475: IC79.7(D3) U$5.13(I/O2)
N$476: IC79.8(D4) U$5.15(I/O3)
N$477: IC79.13(D5) U$5.16(I/O4)
N$478: IC79.14(D6) U$5.17(I/O5)
N$479: IC79.17(D7) U$5.18(I/O6)
N$480: IC79.18(D8) U$5.19(I/O7)
N$481: IC198.2(A:O) IC199.1(A:I0)
N$482: IC61.8(D4) U$11.15(I/O3)
N$483: IC61.13(D5) U$11.16(I/O4)
N$484: IC61.14(D6) U$11.17(I/O5)
N$485: IC61.17(D7) U$11.18(I/O6)
N$486: IC61.18(D8) U$11.19(I/O7)
N$487: IC62.3(D1) U$12.11(I/O0)
N$488: IC62.4(D2) U$12.12(I/O1)
N$489: IC62.7(D3) U$12.13(I/O2)
N$490: IC62.8(D4) U$12.15(I/O3)
N$491: IC62.13(D5) U$12.16(I/O4)
N$492: IC62.14(D6) U$12.17(I/O5)
N$493: IC62.17(D7) U$12.18(I/O6)
N$494: IC62.18(D8) U$12.19(I/O7)
N$495: IC194.6(B:O) IC200.4(B:I0)
N$496: IC200.6(B:O) IC209.4(B:I0)
N$497: IC165.5(2Q) IC215.3(A2)
N$498: IC165.6(3Q) IC215.4(A3)
N$499: IC165.9(4Q) IC215.5(A4)
N$500: IC165.12(5Q) IC215.6(A5)
N$501: IC165.15(6Q) IC215.7(A6)
N$502: IC165.16(7Q) IC215.8(A7)
N$503: IC134.18(D8) U$6.19(I/O7)
N$504: IC134.17(D7) U$6.18(I/O6)
N$505: IC134.14(D6) U$6.17(I/O5)
N$506: IC134.13(D5) U$6.16(I/O4)
N$507: IC134.8(D4) U$6.15(I/O3)
N$508: IC134.7(D3) U$6.13(I/O2)
N$509: IC134.4(D2) U$6.12(I/O1)
N$510: IC134.3(D1) U$6.11(I/O0)
N$511: IC135.3(D1) U$7.11(I/O0)
N$512: IC135.4(D2) U$7.12(I/O1)
N$513: IC135.7(D3) U$7.13(I/O2)
N$514: IC135.8(D4) U$7.15(I/O3)
N$515: IC135.13(D5) U$7.16(I/O4)
N$516: IC135.14(D6) U$7.17(I/O5)
N$517: IC135.17(D7) U$7.18(I/O6)
N$518: IC135.18(D8) U$7.19(I/O7)
N$519: IC136.3(D1) U$8.11(I/O0)
N$520: IC136.4(D2) U$8.12(I/O1)
N$521: IC136.7(D3) U$8.13(I/O2)
N$522: IC136.8(D4) U$8.15(I/O3)
N$523: IC136.13(D5) U$8.16(I/O4)
N$524: IC136.14(D6) U$8.17(I/O5)
N$525: IC136.17(D7) U$8.18(I/O6)
N$526: IC136.18(D8) U$8.19(I/O7)
N$527: IC137.3(D1) U$9.11(I/O0)
N$528: IC54.6(3Q) IC87.4(A3) IC139.4(A3)
N$529: IC54.15(6Q) IC139.7(A6)
N$530: IC251.5(2Q) IC252.3(A2)
N$531: IC54.16(7Q) IC139.8(A7)
N$532: IC54.19(8Q) IC139.9(A8)
N$533: IC137.4(D2) U$9.12(I/O1)
N$534: IC137.7(D3) U$9.13(I/O2)
N$535: IC137.8(D4) U$9.15(I/O3)
N$536: IC137.13(D5) U$9.16(I/O4)
N$537: IC137.14(D6) U$9.17(I/O5)
N$538: IC137.17(D7) U$9.18(I/O6)
N$539: IC137.18(D8) U$9.19(I/O7)
N$540: IC251.6(3Q) IC252.4(A3)
N$541: IC64.1(A:I0) IC152.8(C:O)
N$542: IC165.19(8Q) IC215.9(A8)
N$543: IC246.2(1Q) IC259.2(A1)
N$544: IC246.5(2Q) IC259.3(A2)
N$545: IC246.6(3Q) IC259.4(A3)
N$546: IC246.9(4Q) IC259.5(A4)
N$547: IC246.12(5Q) IC259.6(A5)
N$548: IC54.9(4Q) IC87.5(A4) IC139.5(A4)
N$549: IC246.15(6Q) IC259.7(A6)
N$550: IC246.16(7Q) IC259.8(A7)
N$551: IC246.19(8Q) IC259.9(A8)
N$552: IC217.2(1Q) IC260.2(A1)
N$553: IC217.5(2Q) IC260.3(A2)
N$554: IC217.6(3Q) IC260.4(A3)
N$555: IC217.9(4Q) IC260.5(A4)
N$556: IC217.12(5Q) IC260.6(A5)
N$557: IC217.15(6Q) IC260.7(A6)
N$558: IC217.16(7Q) IC260.8(A7)
N$559: IC217.19(8Q) IC260.9(A8)
N$560: IC262.2(1Q) IC263.2(A1)
N$561: IC262.5(2Q) IC263.3(A2)
N$562: IC262.6(3Q) IC263.4(A3)
N$563: IC262.9(4Q) IC263.5(A4)
N$564: IC77.6(Q3)
N$565: IC262.12(5Q) IC263.6(A5)
N$566: IC262.15(6Q) IC263.7(A6)
N$567: IC70.13(D6) IC81.6(B:O)
N$568: IC77.9(Q4)
N$569: IC18.6(B:O) IC70.12(D7)
N$570: IC262.16(7Q) IC263.8(A7)
N$571: IC77.12(Q5)
N$572: IC262.19(8Q) IC263.9(A8)
N$573: IC261.2(1Q) IC264.2(A1)
N$574: IC17.19(8Q) IC88.10(3B) IC92.9(A8) IC147.1(A:I0)
N$575: IC17.16(7Q) IC88.6(2B) IC92.8(A7)
N$576: IC17.15(6Q) IC88.3(1B) IC92.7(A6)
N$577: IC4.6(3Q) IC111.15(B:A3)
N$578: IC4.9(4Q) IC111.17(B:A4)
N$579: IC4.12(5Q) IC112.11(B:A1)
N$580: IC4.15(6Q) IC112.13(B:A2)
N$581: IC4.16(7Q) IC112.15(B:A3)
N$582: IC4.19(8Q) IC112.17(B:A4)
N$583: IC98.2(1Q) IC113.2(A1)
N$584: IC98.5(2Q) IC113.3(A2)
N$585: IC98.6(3Q) IC113.4(A3)
N$586: IC98.9(4Q) IC113.5(A4)
N$587: IC98.12(5Q) IC113.6(A5)
N$588: IC98.15(6Q) IC113.7(A6)
N$589: IC98.16(7Q) IC113.8(A7)
N$590: IC98.19(8Q) IC113.9(A8)
N$591: IC99.2(1Q) IC114.2(A1)
N$592: IC99.5(2Q) IC114.3(A2)
N$593: IC99.6(3Q) IC114.4(A3)
N$594: IC99.9(4Q) IC114.5(A4)
N$595: IC99.12(5Q) IC114.6(A5)
N$596: IC99.15(6Q) IC114.7(A6)
N$597: IC99.16(7Q) IC114.8(A7)
N$598: IC261.5(2Q) IC264.3(A2)
N$599: IC261.6(3Q) IC264.4(A3)
N$600: IC261.9(4Q) IC264.5(A4)
N$601: IC17.12(5Q) IC90.13(4B) IC92.6(A5)
N$602: IC77.15(Q6)
N$603: IC17.9(4Q) IC90.10(3B) IC92.5(A4)
N$604: IC17.6(3Q) IC90.6(2B) IC92.4(A3)
N$605: IC77.16(Q7)
N$606: IC77.19(Q8)
N$607: IC261.12(5Q) IC264.6(A5)
N$608: IC261.15(6Q) IC264.7(A6)
N$609: IC261.16(7Q) IC264.8(A7)
N$610: IC261.19(8Q) IC264.9(A8)
N$611: IC251.9(4Q) IC252.5(A4)
N$612: IC251.12(5Q) IC252.6(A5)
N$613: IC251.15(6Q) IC252.7(A6)
N$614: IC251.16(7Q) IC252.8(A7)
N$615: IC251.19(8Q) IC252.9(A8)
N$616: IC202.2(1Q) IC253.2(A1)
N$617: IC202.5(2Q) IC253.3(A2)
N$618: IC202.6(3Q) IC253.4(A3)
N$619: IC202.9(4Q) IC253.5(A4)
N$620: IC202.12(5Q) IC253.6(A5)
N$621: IC202.15(6Q) IC253.7(A6)
N$622: IC202.16(7Q) IC253.8(A7)
N$623: IC202.19(8Q) IC253.9(A8)
N$624: IC265.2(1Q) IC266.2(A1)
N$625: IC265.5(2Q) IC266.3(A2)
N$626: IC265.6(3Q) IC266.4(A3)
N$627: IC265.9(4Q) IC266.5(A4)
N$628: IC265.12(5Q) IC266.6(A5)
N$629: IC265.15(6Q) IC266.7(A6)
N$630: IC265.16(7Q) IC266.8(A7)
N$631: IC265.19(8Q) IC266.9(A8)
N$632: IC254.2(1Q) IC267.2(A1)
N$633: IC254.5(2Q) IC267.3(A2)
N$634: IC254.6(3Q) IC267.4(A3)
N$635: IC254.9(4Q) IC267.5(A4)
N$636: IC254.12(5Q) IC267.6(A5)
N$637: IC254.15(6Q) IC267.7(A6)
N$638: IC254.16(7Q) IC267.8(A7)
N$639: IC254.19(8Q) IC267.9(A8)
N$640: IC141.5(B:I2) IC270.4(B:O)
N$641: IC269.2(A:I1) IC271.4(B:O)
N$642: IC273.1(1G) IC273.15(2G) IC274.1(1G) IC274.15(2G) IC275.1(1G) IC275.15(2G) IC276.1(1G) IC276.15(2G) IC279.1(1G) IC279.15(2G) IC280.1(1G) IC280.15(2G) IC281.1(1G) IC281.15(2G) IC282.1(1G) IC282.15(2G)
N$643: IC268.4(1Y) IC285.6(B1)
N$644: IC268.7(2Y) IC285.2(B2)
N$645: IC268.9(3Y) IC285.15(B3)
N$646: IC268.12(4Y) IC285.11(B4)
N$647: IC272.4(1Y) IC283.6(B1)
N$648: IC272.7(2Y) IC283.2(B2)
N$649: IC272.9(3Y) IC283.15(B3)
N$650: IC272.12(4Y) IC283.11(B4)
N$651: IC277.4(1Y) IC284.6(B1)
N$652: IC277.7(2Y) IC284.2(B2)
N$653: IC277.9(3Y) IC284.15(B3)
N$654: IC277.12(4Y) IC284.11(B4)
N$655: IC17.5(2Q) IC90.3(1B) IC92.3(A2)
N$656: IC19.19(8Q) IC86.10(3B) IC91.9(A8)
N$657: IC19.16(7Q) IC86.6(2B) IC91.8(A7)
N$658: IC19.15(6Q) IC86.3(1B) IC91.7(A6)
N$659: IC19.12(5Q) IC89.13(4B) IC91.6(A5)
N$660: IC19.9(4Q) IC89.10(3B) IC91.5(A4)
N$661: IC19.6(3Q) IC89.6(2B) IC91.4(A3)
N$662: IC19.5(2Q) IC89.3(1B) IC91.3(A2)
N$663: IC17.2(1Q) IC86.13(4B) IC92.2(A1)
N$664: IC88.13(4B) IC147.3(A:O)
N$665: IC278.4(1Y) IC286.6(B1)
N$666: IC278.7(2Y) IC286.2(B2)
N$667: IC278.9(3Y) IC286.15(B3)
N$668: IC278.12(4Y) IC286.11(B4)
N$669: IC282.7(1Y) IC283.5(A1)
N$670: IC283.7(C0) IC285.9(C4)
N$671: IC283.9(C4) IC284.7(C0)
N$672: IC284.9(C4) IC286.7(C0)
N$673: IC286.9(C4) IC287.7(C0)
N$674: IC282.9(2Y) IC283.3(A2)
N$675: IC279.7(1Y) IC283.14(A3)
N$676: IC279.9(2Y) IC283.12(A4)
N$677: IC280.7(1Y) IC284.5(A1)
N$678: IC280.9(2Y) IC284.3(A2)
N$679: IC281.7(1Y) IC284.14(A3)
N$680: IC281.9(2Y) IC284.12(A4)
N$681: IC275.7(1Y) IC286.5(A1)
N$682: IC275.9(2Y) IC286.3(A2)
N$683: IC276.7(1Y) IC286.14(A3)
N$684: IC276.9(2Y) IC286.12(A4)
N$685: IC220.1(A:I0) IC222.12(Y3)
N$686: IC273.7(1Y) IC287.5(A1)
N$687: IC222.10(Y5) IC224.1(A:I0)
N$688: IC95.9(C4) IC119.7(C0)
N$689: IC124.9(C4) IC148.7(C0)
N$690: IC95.3(A2) IC161.7(2Y)
N$691: IC95.14(A3) IC161.9(3Y)
N$692: IC95.12(A4) IC161.12(4Y)
N$693: IC119.5(A1) IC196.4(1Y)
N$694: IC119.3(A2) IC196.7(2Y)
N$695: IC119.14(A3) IC196.9(3Y)
N$696: IC119.12(A4) IC196.12(4Y)
N$697: IC124.5(A1) IC211.4(1Y)
N$698: IC124.3(A2) IC211.7(2Y)
N$699: IC124.14(A3) IC211.9(3Y)
N$700: IC124.12(A4) IC211.12(4Y)
N$701: IC148.5(A1) IC212.4(1Y)
N$702: IC148.3(A2) IC212.7(2Y)
N$703: IC148.14(A3) IC212.9(3Y)
N$704: IC148.12(A4) IC212.12(4Y)
N$705: IC229.1(A:I0) IC232.6(B:O)
N$706: IC141.8(C:O) IC232.5(B:I1)
N$707: IC141.11(C:I2) IC233.4(B:O) IC236.10(C:I1)
N$708: IC43.4(B:O) IC45.1(A:I0) IC141.10(C:I1)
N$709: IC236.9(C:I0) IC237.3(A:O)
N$710: IC45.3(A:O) IC238.5(B:I1)
N$711: IC236.11(C:I2) IC238.6(B:O)
N$722: IC273.9(2Y) IC287.3(A2)
N$723: IC274.7(1Y) IC287.14(A3)
N$724: IC274.9(2Y) IC287.12(A4)
N$725: IC288.18(A:Y1)
N$726: IC288.16(A:Y2)
N$727: IC288.14(A:Y3)
N$728: IC288.12(A:Y4)
N$729: IC291.18(A:Y1)
N$730: IC291.16(A:Y2)
N$731: IC291.14(A:Y3)
N$732: IC291.12(A:Y4)
N$733: IC290.18(A:Y1)
N$734: IC290.16(A:Y2)
N$735: IC290.14(A:Y3)
N$736: IC290.12(A:Y4)
N$737: IC288.2(A:A1) IC291.2(A:A1) IC292.2(A:A1) IC301.2(1Q)
N$738: IC288.4(A:A2) IC291.4(A:A2) IC292.4(A:A2) IC301.5(2Q)
N$739: IC288.6(A:A3) IC291.6(A:A3) IC292.6(A:A3) IC301.6(3Q)
N$740: IC288.8(A:A4) IC291.8(A:A4) IC292.8(A:A4) IC301.9(4Q)
N$741: IC289.2(A:A1) IC290.2(A:A1) IC293.2(A:A1) IC301.12(5Q)
N$742: IC289.4(A:A2) IC290.4(A:A2) IC293.4(A:A2) IC301.15(6Q)
N$743: IC289.6(A:A3) IC290.6(A:A3) IC293.6(A:A3) IC301.16(7Q)
N$744: IC289.8(A:A4) IC290.8(A:A4) IC293.8(A:A4) IC301.19(8Q)
N$745: IC292.18(A:Y1)
N$746: IC292.16(A:Y2)
N$747: IC292.14(A:Y3)
N$748: IC292.12(A:Y4)
N$749: IC293.18(A:Y1)
N$750: IC293.16(A:Y2)
N$751: IC293.14(A:Y3)
N$752: IC293.12(A:Y4)
N$753: IC295.2(A:A1) IC296.2(1Q) IC298.2(A:A1) IC299.2(A:A1)
N$754: IC295.4(A:A2) IC296.5(2Q) IC298.4(A:A2) IC299.4(A:A2)
N$755: IC295.6(A:A3) IC296.6(3Q) IC298.6(A:A3) IC299.6(A:A3)
N$756: IC295.8(A:A4) IC296.9(4Q) IC298.8(A:A4) IC299.8(A:A4)
N$757: IC294.2(A:A1) IC296.12(5Q) IC297.2(A:A1) IC300.2(A:A1)
N$758: IC294.4(A:A2) IC296.15(6Q) IC297.4(A:A2) IC300.4(A:A2)
N$759: IC294.6(A:A3) IC296.16(7Q) IC297.6(A:A3) IC300.6(A:A3)
N$760: IC294.8(A:A4) IC296.19(8Q) IC297.8(A:A4) IC300.8(A:A4)
N$761: IC285.4(S1) IC302.2(A1)
N$762: IC285.1(S2) IC302.3(A2)
N$763: IC285.13(S3) IC302.4(A3)
N$764: IC285.10(S4) IC302.5(A4)
N$765: IC283.4(S1) IC302.6(A5)
N$766: IC283.1(S2) IC302.7(A6)
N$767: IC283.13(S3) IC302.8(A7)
N$768: IC283.10(S4) IC302.9(A8)
N$769: IC284.4(S1) IC303.2(A1)
N$770: IC284.1(S2) IC303.3(A2)
N$771: IC284.13(S3) IC303.4(A3)
N$772: IC284.10(S4) IC303.5(A4)
N$773: IC286.4(S1) IC303.6(A5)
N$774: IC286.1(S2) IC303.7(A6)
N$775: IC286.13(S3) IC303.8(A7)
N$776: IC286.10(S4) IC303.9(A8)
N$777: IC28.2(A1) IC287.4(S1)
N$778: IC28.3(A2) IC287.1(S2)
N$779: IC28.4(A3) IC287.13(S3)
N$780: IC28.5(A4) IC287.10(S4)
N$781: IC54.12(5Q) IC87.6(A5) IC139.6(A5)
N$1062: IC411.3(A:S2) R23.1 S3.1(O)
N$1063: IC411.1(A:R) R24.1 S3.3(S)
N$1067: IC410.3(B:I) IC412.3(Q1)
N$1068: IC412.7(CLK) IC413.3(A:CLK) SW1.C
N$1069: IC412.1(M) IC412.2(N) IC415.6(B:O)
N$1218: IC29.2(A1) IC44.2(A1) IC544.2(1Q)
N$1219: IC29.3(A2) IC44.3(A2) IC544.5(2Q)
N$1220: IC29.4(A3) IC44.4(A3) IC544.6(3Q)
N$1222: IC44.7(A6) IC544.15(6Q)
N$1223: IC44.8(A7) IC544.16(7Q)
N$1224: IC44.9(A8) IC544.19(8Q)
N$1560: IC29.5(A4) IC44.5(A4) IC544.9(4Q)
NORMAL_CLK: SW1.2
NOT_CONDITION: IC74.4(B:I0)
NOT_RST: IC75.1(CLR) IC76.1(CLR) IC77.1(CLR) IC78.1(CLR) IC79.1(CLR) IC134.1(CLR) IC135.1(CLR) IC136.1(CLR) IC137.1(CLR)
OF: IC122.5(A4) IC156.10(2C0) IC227.9(Q4) IC256.6(1C0)
OF_FROM_ALU: IC126.8(4D) IC156.12(2C2) IC256.5(1C1)
OF_IN_SRC_0: IC256.14(A)
OF_IN_SRC_1: IC256.2(B)
PANEL_MEM_IO: RN4.3
PANEL_RD: RN4.1
PANEL_WR: RN4.2
PC_H_0: IC211.2(1A) IC277.3(1B)
PC_H_1: IC211.5(2A) IC277.6(2B)
PC_H_2: IC211.11(3A) IC277.10(3B)
PC_H_3: IC211.14(4A) IC277.13(4B)
PC_H_4: IC212.2(1A) IC278.3(1B)
PC_H_5: IC212.5(2A) IC278.6(2B)
PC_H_6: IC212.11(3A) IC278.10(3B)
PC_H_7: IC212.14(4A) IC278.13(4B)
PC_H_OUT: IC107.19(B:G) IC108.19(B:G)
PC_H_WRT: IC6.1(G)
PC_IN_SRC: IC96.1(!A!/B) IC97.1(!A!/B) IC103.1(!A!/B) IC104.1(!A!/B)
PC_L_0: IC161.2(1A) IC268.3(1B)
PC_L_1: IC161.5(2A) IC268.6(2B)
PC_L_2: IC161.11(3A) IC268.10(3B)
PC_L_3: IC161.14(4A) IC268.13(4B)
PC_L_4: IC196.2(1A) IC272.3(1B)
PC_L_5: IC196.5(2A) IC272.6(2B)
PC_L_6: IC196.11(3A) IC272.10(3B)
PC_L_7: IC196.14(4A) IC272.13(4B)
PC_L_OUT: IC105.19(B:G) IC106.19(B:G)
PC_L_WRT: IC48.1(G)
PC_MAR_ADDER_OUT_0: IC48.3(1D) IC96.4(1Y)
PC_MAR_ADDER_OUT_1: IC48.4(2D) IC96.7(2Y)
PC_MAR_ADDER_OUT_15: IC6.18(8D) IC104.12(4Y)
PCH_0: IC6.2(1Q) IC107.11(B:A1)
PCH_1: IC6.5(2Q) IC107.13(B:A2)
PCH_2: IC6.6(3Q) IC107.15(B:A3)
PCH_3: IC6.9(4Q) IC107.17(B:A4)
PCH_4: IC6.12(5Q) IC108.11(B:A1)
PCH_5: IC6.15(6Q) IC108.13(B:A2)
PCH_6: IC6.16(7Q) IC108.15(B:A3)
PCH_7: IC6.19(8Q) IC108.17(B:A4)
PCL_0: IC48.2(1Q) IC105.11(B:A1)
PCL_1: IC48.5(2Q) IC105.13(B:A2)
PCL_2: IC48.6(3Q) IC105.15(B:A3)
PCL_3: IC48.9(4Q) IC105.17(B:A4)
PCL_4: IC48.12(5Q) IC106.11(B:A1)
PCL_5: IC48.15(6Q) IC106.13(B:A2)
PCL_6: IC48.16(7Q) IC106.15(B:A3)
PCL_7: IC48.19(8Q) IC106.17(B:A4)
PF: IC70.15(D4) IC122.6(A5) IC208.6(1C0) IC227.12(Q5)
PF_FROM_ALU: IC59.2(A:O) IC208.5(1C1)
PF_IN_SRC_0: IC208.14(A)
PF_IN_SRC_1: IC208.2(B)
PROG_MODE: IC250.5(B:I1)
RD: IC60.2(Q1) IC69.11(B:A1)
REQ_ENCOD_0: IC222.1(A)
REQ_ENCOD_1: IC154.6(A5) IC222.2(B) IC226.7(A1)
REQ_ENCOD_2: IC154.5(A4) IC222.3(C) IC226.6(A2)
RST: IC128.15(CLR) IC144.15(CLR) IC248.15(CLR) IC249.15(CLR) IC412.15(CLR) IC414.3(B:I) R25.1 S5.2(P)
SF: IC122.4(A3) IC156.6(1C0) IC227.6(Q3) IC255.6(1C0)
SF_FROM_ALU: IC126.7(3D) IC156.4(1C2)
SF_IN_SRC_0: IC255.14(A)
SF_IN_SRC_1: IC255.2(B)
SF_XOR_OF: IC70.14(D5) IC72.6(B:O) IC81.4(B:I0)
SHR_MACHINE_H_OUT: IC92.1(G1) IC92.19(G2)
SHR_MACHINE_H_WRT: IC17.1(G)
SHR_MACHINE_IN_SRC: IC86.1(!A!/B) IC88.1(!A!/B) IC89.1(!A!/B) IC90.1(!A!/B)
SHR_MACHINE_L_OUT: IC91.1(G1) IC91.19(G2)
SHR_MACHINE_L_WRT: IC19.1(G)
SHR_MACHINE_TYPE: IC147.2(A:I1)
SI_H_OUT: IC253.1(G1) IC253.19(G2)
SI_H_WRT: IC202.1(G)
SI_L_OUT: IC252.1(G1) IC252.19(G2)
SI_L_WRT: IC251.1(G)
SINGLE_STEP_CLK: IC411.4(A:Q) SW1.1
SPH_OUT: IC111.19(B:G) IC112.19(B:G)
SPH_WRT: IC4.1(G)
SPL_OUT: IC109.19(B:G) IC110.19(B:G)
SPL_WRT: IC5.1(G)
SS_H_0: IC275.4(1C2)
SS_H_1: IC275.12(2C2)
SS_H_2: IC276.4(1C2)
SS_H_3: IC276.12(2C2)
SS_H_4: IC273.4(1C2)
SS_H_5: IC273.12(2C2)
SS_H_6: IC274.4(1C2)
SS_H_7: IC274.12(2C2)
SS_H_OUT: IC260.1(G1) IC260.19(G2)
SS_H_WRT: IC217.1(G)
SS_L_0: IC282.4(1C2)
SS_L_1: IC282.12(2C2)
SS_L_2: IC279.4(1C2)
SS_L_3: IC279.12(2C2)
SS_L_4: IC280.4(1C2)
SS_L_5: IC280.12(2C2)
SS_L_6: IC281.4(1C2)
SS_L_7: IC281.12(2C2)
SS_L_OUT: IC259.1(G1) IC259.19(G2)
SS_L_WRT: IC246.1(G)
STOP_CLK: IC413.2(A:D) IC413.5(A:Q) IC415.4(B:I0) R26.1 S6.2(P)
TDR0_L_WRT: IC54.1(G) IC544.1(G)
TDR_H_X_OUT: IC87.1(G1) IC87.19(G2)
TDR_H_Y_OUT: IC139.1(G1) IC139.19(G2)
TDR_L_X_OUT: IC29.1(G1) IC29.19(G2)
TDR_L_Y_OUT: IC44.1(G1) IC44.19(G2)
TRAP_ACK: IC94.3(B:I)
TRAP_PENDING: IC47.3(A:O) IC232.4(B:I0) IC233.3(B:I) IC235.11(C:I2)
TRAP_REQ: IC39.3(A:CLK) IC47.1(A:I0) R1.2
TRISTATE: IC28.1(G1) IC28.19(G2) IC69.19(B:G) IC250.6(B:O) IC302.1(G1) IC302.19(G2) IC303.1(G1) IC303.19(G2)
TYP0: IC214.5(B:I1) IC230.3(B:I)
TYP1: IC213.2(A:I1) IC231.3(B:I) IC235.9(C:I0) IC237.1(A:I0)
TYP_0: IC85.1(A:I0)
TYP_1: IC84.3(B:I)
U_AD0: IC32.2(Q1) U$6.10(A0) U$7.10(A0) U$8.10(A0) U$9.10(A0)
U_AD1: IC32.5(Q2) U$6.9(A1) U$7.9(A1) U$8.9(A1) U$9.9(A1)
U_AD2: IC32.6(Q3) U$6.8(A2) U$7.8(A2) U$8.8(A2) U$9.8(A2)
U_AD3: IC32.9(Q4) U$6.7(A3) U$7.7(A3) U$8.7(A3) U$9.7(A3)
U_AD4: IC32.12(Q5) U$6.6(A4) U$7.6(A4) U$8.6(A4) U$9.6(A4)
U_AD5: IC32.15(Q6) U$6.5(A5) U$7.5(A5) U$8.5(A5) U$9.5(A5)
U_AD6: IC32.16(Q7) U$6.4(A6) U$7.4(A6) U$8.4(A6) U$9.4(A6)
U_AD7: IC32.19(Q8) U$6.3(A7) U$7.3(A7) U$8.3(A7) U$9.3(A7)
U_AD8: IC33.2(Q1) U$6.25(A8) U$7.25(A8) U$8.25(A8) U$9.25(A8)
U_AD9: IC33.5(Q2) U$6.24(A9) U$7.24(A9) U$8.24(A9) U$9.24(A9)
U_AD10: IC33.6(Q3) U$6.21(A10) U$7.21(A10) U$8.21(A10) U$9.21(A10)
U_AD11: IC33.9(Q4) U$6.23(A11) U$7.23(A11) U$8.23(A11) U$9.23(A11)
U_AD12: IC33.12(Q5) U$6.2(A12) U$7.2(A12) U$8.2(A12) U$9.2(A12)
U_AD13: IC33.15(Q6) U$6.26(A13) U$7.26(A13) U$8.26(A13) U$9.26(A13)
U_AD14: IC33.16(Q7) IC53.14(A3)
U_AD15: IC33.19(Q8) IC53.12(A4)
U_AD_BUFF0: U$1.10(A0)
U_AD_BUFF1: U$1.9(A1)
U_AD_BUFF2: U$1.8(A2)
U_AD_BUFF3: U$1.7(A3)
U_AD_BUFF4: U$1.6(A4)
U_AD_BUFF5: U$1.5(A5)
U_AD_BUFF6: U$1.4(A6)
U_AD_BUFF7: U$1.3(A7)
U_AD_BUFF8: U$1.25(A8)
U_AD_BUFF9: U$1.24(A9)
U_AD_BUFF10: U$1.21(A10)
U_AD_BUFF11: U$1.23(A11)
U_AD_BUFF12: U$1.2(A12)
U_AD_BUFF13: U$1.26(A13)
U_ADDER_0: IC50.4(S1) IC186.4(D0)
U_ADDER_1: IC160.4(D0)
U_ADDER_2: IC159.4(D0)
U_ADDER_3: IC142.4(D0)
U_ADDER_4: IC129.4(D0)
U_ADDER_5: IC73.4(D0)
U_ADDER_6: IC34.4(D0)
U_ADDER_7: IC35.4(D0)
U_ADDER_8: IC36.4(D0)
U_ADDER_9: IC37.4(D0)
U_ADDER_10: IC38.4(D0)
U_ADDER_11: IC40.4(D0)
U_ADDER_12: IC41.4(D0)
U_ADDER_13: IC53.1(S2) IC71.4(D0)
U_ADDER_14: IC20.4(D0)
U_ADDER_15: IC172.4(D0)
U_CF: IC126.5(2Q) IC155.11(2C1) IC167.3(1B)
U_DMA_0: IC186.15(D4)
U_DMA_1: IC160.15(D4)
U_DMA_2: IC159.15(D4)
U_DMA_3: IC142.15(D4)
U_DMA_4: IC129.15(D4)
U_DMA_5: IC73.15(D4)
U_DMA_6: IC34.15(D4)
U_DMA_7: IC35.15(D4)
U_DMA_8: IC36.15(D4)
